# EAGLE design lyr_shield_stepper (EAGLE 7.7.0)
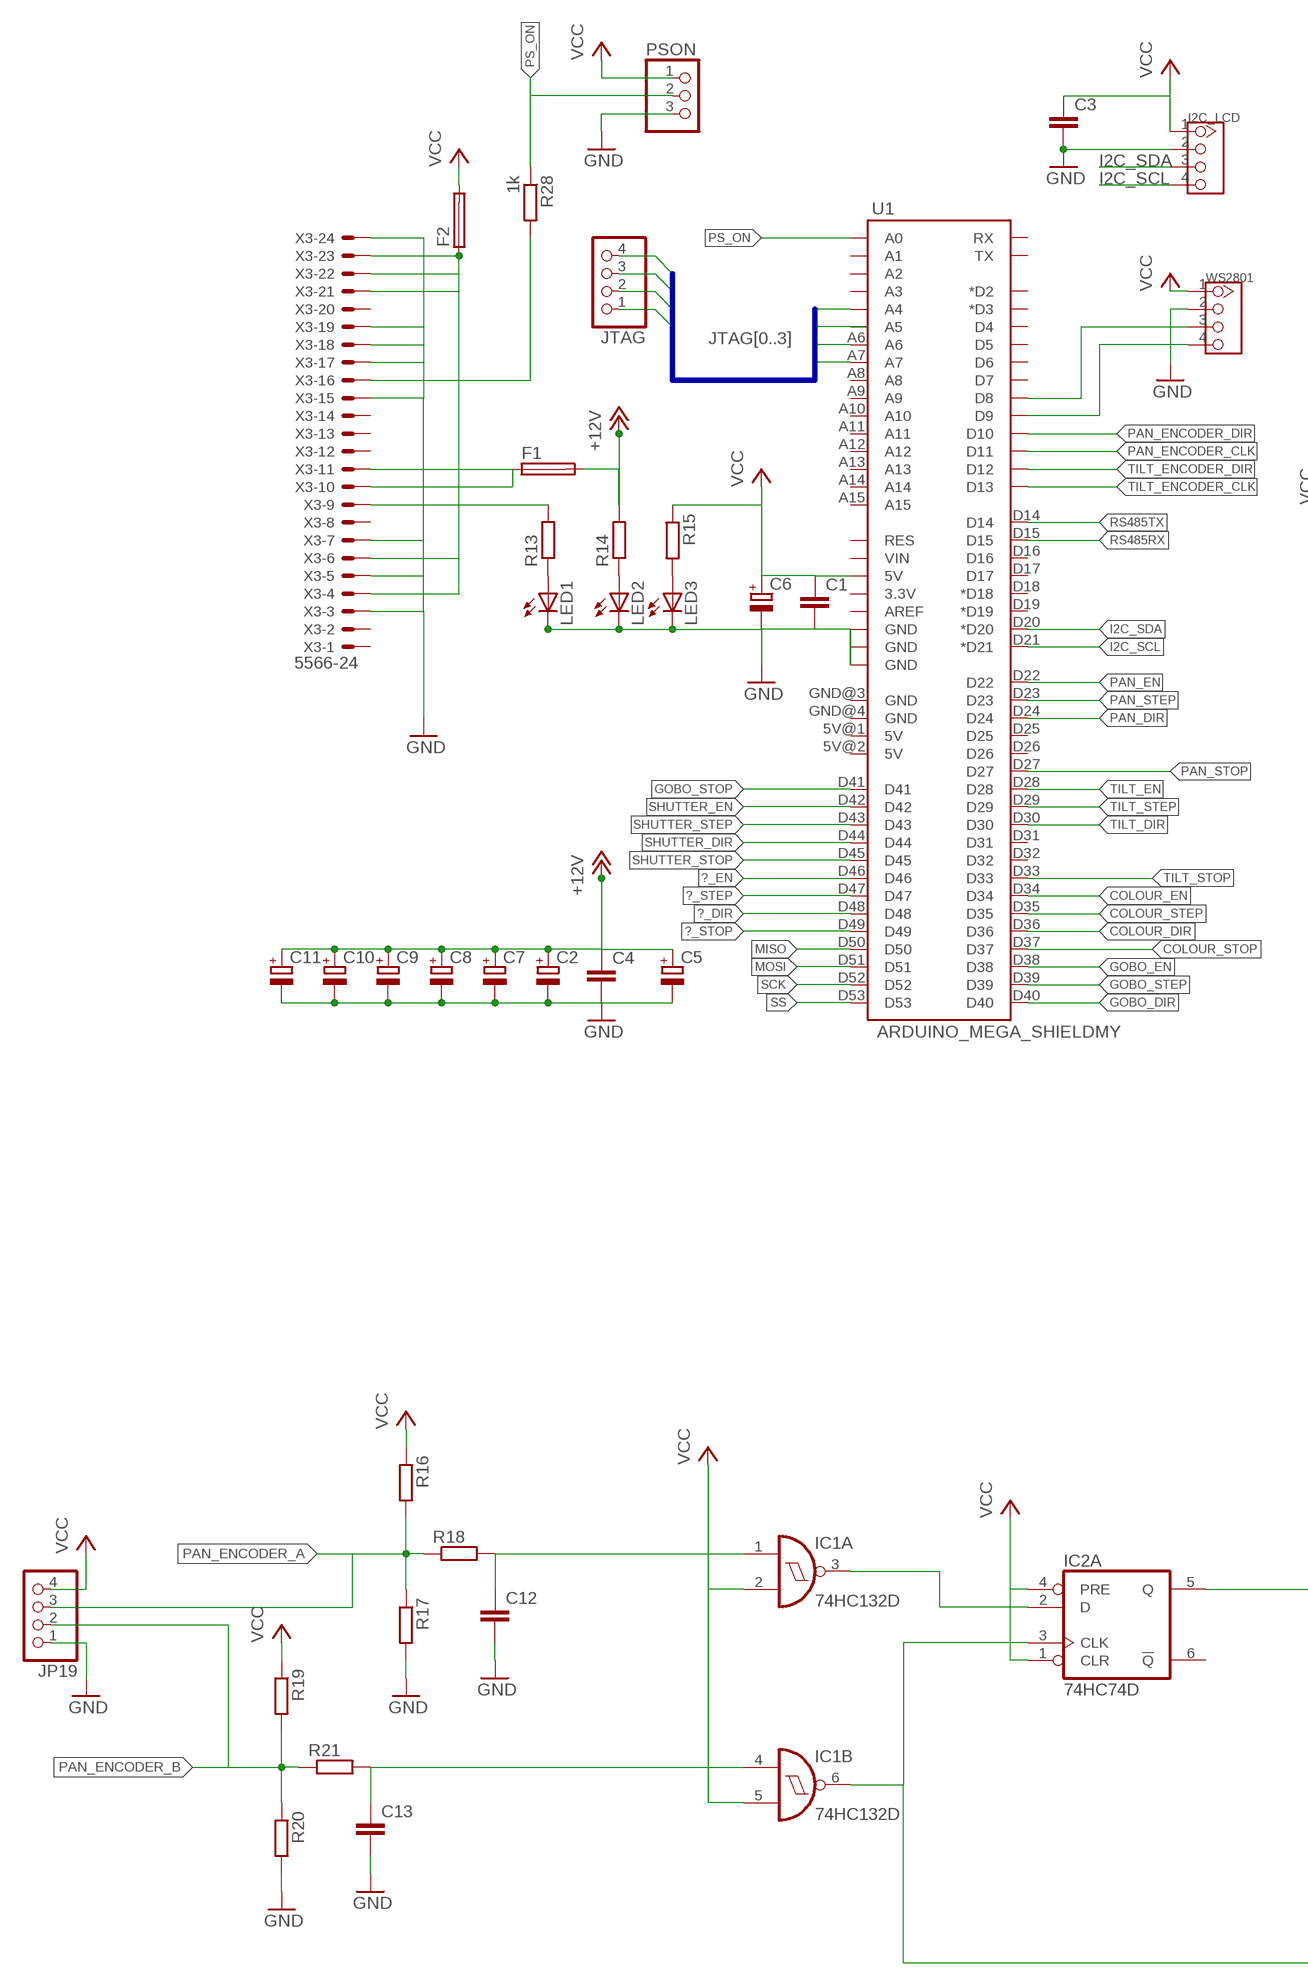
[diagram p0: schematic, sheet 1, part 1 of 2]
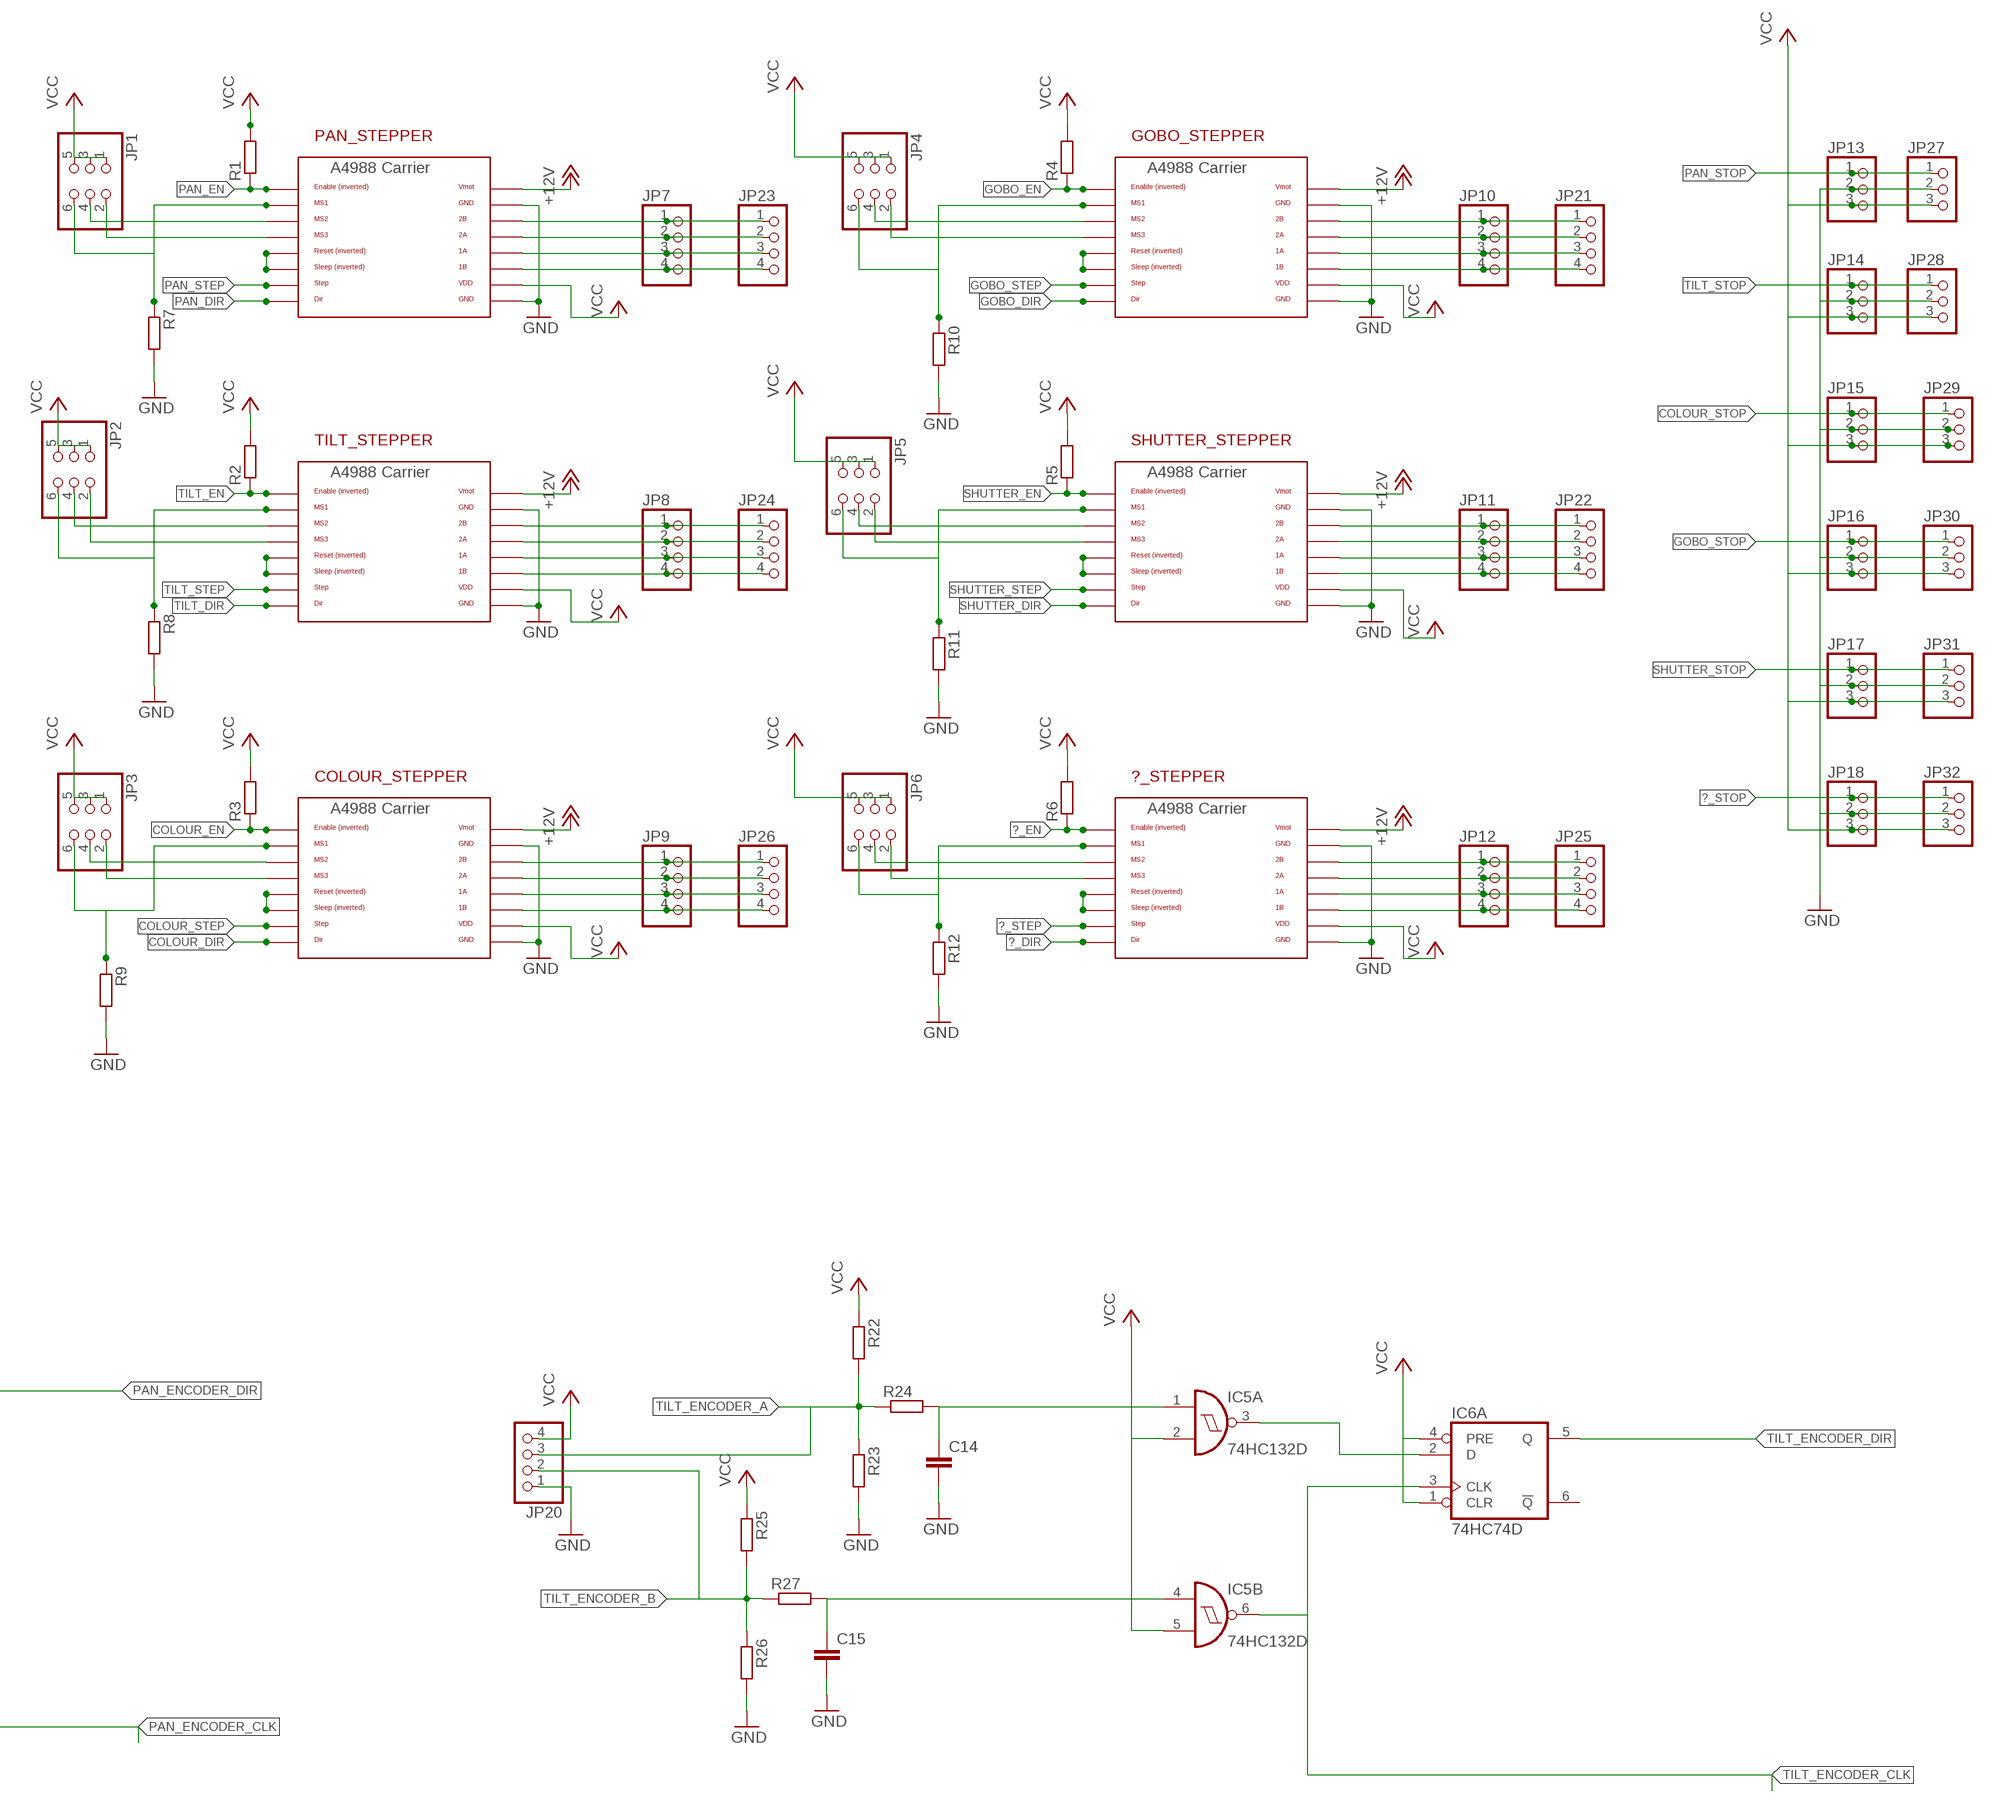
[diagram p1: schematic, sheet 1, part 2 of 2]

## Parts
?_STEPPER  POLOLU_A4983CARRIER  [A4988BREAKOUT]
C1  C-EU025-025X050  [C025-025X050]
C2  CPOL-EUE1.8-4  [E1,8-4]
C3  C-EU025-025X050  [C025-025X050]
C4  C-EU050-025X075  [C050-025X075]
C5  CPOL-EUE5-8.5  [E5-8,5]
C6  CPOL-EUE5-8.5  [E5-8,5]
C7  CPOL-EUE1.8-4  [E1,8-4]
C8  CPOL-EUE1.8-4  [E1,8-4]
C9  CPOL-EUE1.8-4  [E1,8-4]
C10  CPOL-EUE1.8-4  [E1,8-4]
C11  CPOL-EUE1.8-4  [E1,8-4]
C12  C-EU025-025X050  [C025-025X050]
C13  C-EU025-025X050  [C025-025X050]
C14  C-EU025-025X050  [C025-025X050]
C15  C-EU025-025X050  [C025-025X050]
COLOUR_STEPPER  POLOLU_A4983CARRIER  [A4988BREAKOUT]
F1  PTCFUSE  [LITTLEFUSE]
F2  PTCFUSE  [LITTLEFUSE]
GOBO_STEPPER  POLOLU_A4983CARRIER  [A4988BREAKOUT]
I2C_LCD  CONNECTOR_TWIG-4P-2.090D  [CONNECTOR_4P-2.0-90D]
IC1  74HC132D  [SO14]
IC2  74HC74D  [SO14]
IC5  74HC132D  [SO14]
IC6  74HC74D  [SO14]
JP1  PINHD-2X3  [2X03]
JP2  PINHD-2X3  [2X03]
JP3  PINHD-2X3  [2X03]
JP4  PINHD-2X3  [2X03]
JP5  PINHD-2X3  [2X03]
JP6  PINHD-2X3  [2X03]
JP7  PINHD-1X4  [1X04]
JP8  PINHD-1X4  [1X04]
JP9  PINHD-1X4  [1X04]
JP10  PINHD-1X4  [1X04]
JP11  PINHD-1X4  [1X04]
JP12  PINHD-1X4  [1X04]
JP13  PINHD-1X3  [1X03]
JP14  PINHD-1X3  [1X03]
JP15  PINHD-1X3  [1X03]
JP16  PINHD-1X3  [1X03]
JP17  PINHD-1X3  [1X03]
JP18  PINHD-1X3  [1X03]
JP19  PINHD-1X4  [1X04]
JP20  PINHD-1X4  [1X04]
JP21  PINHD-1X4  [1X04]
JP22  PINHD-1X4  [1X04]
JP23  PINHD-1X4  [1X04]
JP24  PINHD-1X4  [1X04]
JP25  PINHD-1X4  [1X04]
JP26  PINHD-1X4  [1X04]
JP27  PINHD-1X3  [1X03]
JP28  PINHD-1X3  [1X03]
JP29  PINHD-1X3  [1X03]
JP30  PINHD-1X3  [1X03]
JP31  PINHD-1X3  [1X03]
JP32  PINHD-1X3  [1X03]
JTAG  PINHD-1X4  [1X04]
LED1  LED5MM  [LED5MM]
LED2  LED5MM  [LED5MM]
LED3  LED5MM  [LED5MM]
PAN_STEPPER  POLOLU_A4983CARRIER  [A4988BREAKOUT]
PSON  PINHD-1X3  [1X03]
R1  R-EU_0207/7  [0207/7]
R2  R-EU_0207/7  [0207/7]
R3  R-EU_0207/7  [0207/7]
R4  R-EU_0207/7  [0207/7]
R5  R-EU_0207/7  [0207/7]
R6  R-EU_0207/7  [0207/7]
R7  R-EU_0207/7  [0207/7]
R8  R-EU_0207/7  [0207/7]
R9  R-EU_0207/7  [0207/7]
R10  R-EU_0207/7  [0207/7]
R11  R-EU_0207/7  [0207/7]
R12  R-EU_0207/7  [0207/7]
R13  R-EU_0207/2V  [0207/2V]
R14  R-EU_0207/2V  [0207/2V]
R15  R-EU_0207/2V  [0207/2V]
R16  R-EU_0207/7  [0207/7]
R17  R-EU_0207/7  [0207/7]
R18  R-EU_0207/7  [0207/7]
R19  R-EU_0207/7  [0207/7]
R20  R-EU_0207/7  [0207/7]
R21  R-EU_0207/7  [0207/7]
R22  R-EU_0207/7  [0207/7]
R23  R-EU_0207/7  [0207/7]
R24  R-EU_0207/7  [0207/7]
R25  R-EU_0207/7  [0207/7]
R26  R-EU_0207/7  [0207/7]
R27  R-EU_0207/7  [0207/7]
R28  1k  R-EU_0207/7  [0207/7]
SHUTTER_STEPPER  POLOLU_A4983CARRIER  [A4988BREAKOUT]
TILT_STEPPER  POLOLU_A4983CARRIER  [A4988BREAKOUT]
U1  ARDUINO_MEGA_SHIELDMY  [MY_ARDUINO_MEGA_SHIELD]
WS2801  CONNECTOR_TWIG-4P-2.090D  [CONNECTOR_4P-2.0-90D]
X3  5566-24  [5566-24]

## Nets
+12V [vcc]: ?_STEPPER.VMOT C2.+ C4.1 C5.+ C7.+ C8.+ C9.+ C10.+ C11.+ COLOUR_STEPPER.VMOT F1.2 GOBO_STEPPER.VMOT PAN_STEPPER.VMOT R14.2 SHUTTER_STEPPER.VMOT TILT_STEPPER.VMOT
?_DIR: ?_STEPPER.DIR U1.D48
?_EN: ?_STEPPER.EN R6.1 U1.D46
?_STEP: ?_STEPPER.STEP U1.D47
?_STOP: JP18.1 JP32.1 U1.D49
COLOUR_DIR: COLOUR_STEPPER.DIR U1.D36
COLOUR_EN: COLOUR_STEPPER.EN R3.1 U1.D34
COLOUR_STEP: COLOUR_STEPPER.STEP U1.D35
COLOUR_STOP: JP15.1 JP29.1 U1.D37
GND [gnd]: ?_STEPPER.GND ?_STEPPER.GND@0(GND) C1.2 C2.- C3.2 C4.2 C5.- C6.- C7.- C8.- C9.- C10.- C11.- C12.2 C13.2 C14.2 C15.2 COLOUR_STEPPER.GND COLOUR_STEPPER.GND@0(GND) GOBO_STEPPER.GND GOBO_STEPPER.GND@0(GND) I2C_LCD.2 JP13.2 JP14.2 JP15.2 JP16.2 JP17.2 JP18.2 JP19.1 JP20.1 JP27.2 JP28.2 JP29.2 JP30.2 JP31.2 JP32.2 LED1.K(C) LED2.K(C) LED3.K(C) PAN_STEPPER.GND PAN_STEPPER.GND@0(GND) PSON.3 R7.2 R8.2 R9.2 R10.2 R11.2 R12.2 R17.2 R20.2 R23.2 R26.2 SHUTTER_STEPPER.GND SHUTTER_STEPPER.GND@0(GND) TILT_STEPPER.GND TILT_STEPPER.GND@0(GND) U1.GND@0(GND) U1.GND@1(GND) U1.GND@2(GND) WS2801.2 X3.3 X3.5 X3.7 X3.15 X3.17 X3.18 X3.19 X3.24
GOBO_DIR: GOBO_STEPPER.DIR U1.D40
GOBO_EN: GOBO_STEPPER.EN R4.1 U1.D38
GOBO_STEP: GOBO_STEPPER.STEP U1.D39
GOBO_STOP: JP16.1 JP30.1 U1.D41
I2C_SCL: I2C_LCD.4 U1.D21(*D21)
I2C_SDA: I2C_LCD.3 U1.D20(*D20)
JTAG0: JTAG.1 U1.A4
JTAG1: JTAG.2
JTAG2: JTAG.3 U1.A6
JTAG3: JTAG.4 U1.A7
MISO: U1.D50
MOSI: U1.D51
N$1: PAN_STEPPER.RST PAN_STEPPER.SLP(SLEEP)
N$2: TILT_STEPPER.RST TILT_STEPPER.SLP(SLEEP)
N$3: COLOUR_STEPPER.RST COLOUR_STEPPER.SLP(SLEEP)
N$4: GOBO_STEPPER.RST GOBO_STEPPER.SLP(SLEEP)
N$5: SHUTTER_STEPPER.RST SHUTTER_STEPPER.SLP(SLEEP)
N$6: ?_STEPPER.RST ?_STEPPER.SLP(SLEEP)
N$7: JP1.6 PAN_STEPPER.MS1 R7.1
N$8: JP1.2 PAN_STEPPER.MS3
N$9: JP1.4 PAN_STEPPER.MS2
N$10: JP2.6 R8.1 TILT_STEPPER.MS1
N$11: JP2.2 TILT_STEPPER.MS3
N$12: JP2.4 TILT_STEPPER.MS2
N$13: COLOUR_STEPPER.MS1 JP3.6 R9.1
N$14: COLOUR_STEPPER.MS3 JP3.2
N$15: COLOUR_STEPPER.MS2 JP3.4
N$16: GOBO_STEPPER.MS1 JP4.6 R10.1
N$17: GOBO_STEPPER.MS3 JP4.2
N$18: GOBO_STEPPER.MS2 JP4.4
N$19: JP5.6 R11.1 SHUTTER_STEPPER.MS1
N$20: JP5.2 SHUTTER_STEPPER.MS3
N$21: JP5.4 SHUTTER_STEPPER.MS2
N$22: ?_STEPPER.MS1 JP6.6 R12.1
N$23: ?_STEPPER.MS3 JP6.2
N$24: ?_STEPPER.MS2 JP6.4
N$25 [vcc]: JP7.1 JP23.1 PAN_STEPPER.2B
N$26 [vcc]: JP7.2 JP23.2 PAN_STEPPER.2A
N$27 [vcc]: JP7.3 JP23.3 PAN_STEPPER.1A
N$28: IC1.3(A:O) IC2.2(A:D)
N$29: C12.1 IC1.1(A:I0) R18.2
N$30: R28.2 X3.16
N$31 [vcc]: JP7.4 JP23.4 PAN_STEPPER.1B
N$32 [vcc]: JP8.1 JP24.1 TILT_STEPPER.2B
N$33 [vcc]: JP8.2 JP24.2 TILT_STEPPER.2A
N$34 [vcc]: JP8.3 JP24.3 TILT_STEPPER.1A
N$35 [vcc]: JP8.4 JP24.4 TILT_STEPPER.1B
N$36 [vcc]: COLOUR_STEPPER.2B JP9.1 JP26.1
N$37 [vcc]: COLOUR_STEPPER.2A JP9.2 JP26.2
N$38 [vcc]: COLOUR_STEPPER.1A JP9.3 JP26.3
N$39 [vcc]: COLOUR_STEPPER.1B JP9.4 JP26.4
N$40 [vcc]: GOBO_STEPPER.2B JP10.1 JP21.1
N$41 [vcc]: GOBO_STEPPER.2A JP10.2 JP21.2
N$42 [vcc]: GOBO_STEPPER.1A JP10.3 JP21.3
N$43 [vcc]: GOBO_STEPPER.1B JP10.4 JP21.4
N$44 [vcc]: JP11.1 JP22.1 SHUTTER_STEPPER.2B
N$45 [vcc]: JP11.2 JP22.2 SHUTTER_STEPPER.2A
N$46 [vcc]: JP11.3 JP22.3 SHUTTER_STEPPER.1A
N$47 [vcc]: JP11.4 JP22.4 SHUTTER_STEPPER.1B
N$48 [vcc]: ?_STEPPER.2B JP12.1 JP25.1
N$49 [vcc]: ?_STEPPER.2A JP12.2 JP25.2
N$50 [vcc]: ?_STEPPER.1A JP12.3 JP25.3
N$51 [vcc]: ?_STEPPER.1B JP12.4 JP25.4
N$52: LED1.A R13.1
N$53: U1.D8 WS2801.3
N$54: R13.2 X3.9
N$55: LED3.A R15.2
N$56: LED2.A R14.1
N$57: U1.D9 WS2801.4
N$58 [vcc]: F1.1 X3.10 X3.11
N$60 [vcc]: F2.1 X3.4 X3.6 X3.21 X3.22 X3.23
N$61: C13.1 IC1.4(B:I0) R21.2
N$62: IC5.3(A:O) IC6.2(A:D)
N$63: C14.1 IC5.1(A:I0) R24.2
N$64: C15.1 IC5.4(B:I0) R27.2
PAN_DIR: PAN_STEPPER.DIR U1.D24
PAN_EN: PAN_STEPPER.EN R1.1 U1.D22
PAN_ENCODER_A: JP19.3 R16.2 R17.1 R18.1
PAN_ENCODER_B: JP19.2 R19.2 R20.1 R21.1
PAN_ENCODER_CLK: IC1.6(B:O) IC2.3(A:CLK)
PAN_ENCODER_DIR: IC2.5(A:Q)
PAN_STEP: PAN_STEPPER.STEP U1.D23
PAN_STOP: JP13.1 JP27.1 U1.D27
PS_ON: PSON.2 R28.1
RS485RX: U1.D15
RS485TX: U1.D14
SCK: U1.D52
SHUTTER_DIR: SHUTTER_STEPPER.DIR U1.D44
SHUTTER_EN: R5.1 SHUTTER_STEPPER.EN U1.D42
SHUTTER_STEP: SHUTTER_STEPPER.STEP U1.D43
SHUTTER_STOP: JP17.1 JP31.1 U1.D45
SS: U1.D53
TILT_DIR: TILT_STEPPER.DIR U1.D30
TILT_EN: R2.1 TILT_STEPPER.EN U1.D28
TILT_ENCODER_A: JP20.3 R22.2 R23.1 R24.1
TILT_ENCODER_B: JP20.2 R25.2 R26.1 R27.1
TILT_ENCODER_CLK: IC5.6(B:O) IC6.3(A:CLK)
TILT_ENCODER_DIR: IC6.5(A:Q)
TILT_STEP: TILT_STEPPER.STEP U1.D29
TILT_STOP: JP14.1 JP28.1 U1.D33
VCC [vcc]: ?_STEPPER.VDD C1.1 C3.1 C6.+ COLOUR_STEPPER.VDD F2.2 GOBO_STEPPER.VDD I2C_LCD.1 IC1.2(A:I1) IC1.5(B:I1) IC2.1(A:CLR) IC2.4(A:PRE) IC5.2(A:I1) IC5.5(B:I1) IC6.1(A:CLR) IC6.4(A:PRE) JP1.1 JP1.3 JP1.5 JP2.1 JP2.3 JP2.5 JP3.1 JP3.3 JP3.5 JP4.1 JP4.3 JP4.5 JP5.1 JP5.3 JP5.5 JP6.1 JP6.3 JP6.5 JP13.3 JP14.3 JP15.3 JP16.3 JP17.3 JP18.3 JP19.4 JP20.4 JP27.3 JP28.3 JP29.3 JP30.3 JP31.3 JP32.3 PAN_STEPPER.VDD PSON.1 R1.2 R2.2 R3.2 R4.2 R5.2 R6.2 R15.1 R16.1 R19.1 R22.1 R25.1 SHUTTER_STEPPER.VDD TILT_STEPPER.VDD U1.5V@0(5V) WS2801.1
Unconnected: IC1.8(C:O) IC1.9(C:I0) IC1.10(C:I1) IC1.11(D:O) IC1.12(D:I0) IC1.13(D:I1) IC2.6(A:!Q) IC2.8(B:!Q) IC2.9(B:Q) IC2.10(B:PRE) IC2.11(B:CLK) IC2.12(B:D) IC2.13(B:CLR) IC5.8(C:O) IC5.9(C:I0) IC5.10(C:I1) IC5.11(D:O) IC5.12(D:I0) IC5.13(D:I1) IC6.6(A:!Q) IC6.8(B:!Q) IC6.9(B:Q) IC6.10(B:PRE) IC6.11(B:CLK) IC6.12(B:D) IC6.13(B:CLR) U1.3.3V U1.5V@1(5V) U1.5V@2(5V) U1.A0 U1.A1 U1.A2 U1.A3 U1.A5 U1.A8 U1.A9 U1.A10 U1.A11 U1.A12 U1.A13 U1.A14 U1.A15 U1.AREF U1.D2(*D2) U1.D3(*D3) U1.D4 U1.D5 U1.D6 U1.D7 U1.D10 U1.D11 U1.D12 U1.D13 U1.D16 U1.D17 U1.D18(*D18) U1.D19(*D19) U1.D25 U1.D26 U1.D31 U1.D32 U1.GND@3(GND) U1.GND@4(GND) U1.RES U1.RX U1.TX U1.VIN X3.1 X3.2 X3.8 X3.12 X3.13 X3.14 X3.20

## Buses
JTAG[0..3]

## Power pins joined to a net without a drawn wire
GND: IC1.7(P:GND) IC2.7(P:GND) IC5.7(P:GND) IC6.7(P:GND)
VCC: IC1.14(P:VCC) IC2.14(P:VCC) IC5.14(P:VCC) IC6.14(P:VCC)

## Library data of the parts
?_STEPPER COLOUR_STEPPER GOBO_STEPPER PAN_STEPPER SHUTTER_STEPPER TILT_STEPPER = lyr_shield_stepper:POLOLU_A4983CARRIER
C1 C3 C4 C12-C15 = rcl:C-EU: CAPACITOR, European symbol
C2 C5-C11 = rcl:CPOL-EU: POLARIZED CAPACITOR, European symbol
F1 F2 = RepRapjr:PTCFUSE: LITTLEFUSE
I2C_LCD WS2801 = lyr_shield_stepper:CONNECTOR_TWIG-4P-2.0
IC1 IC5 = 74xx-eu:74*132: Quad 2-input NAND schmitt trigger
IC2 IC6 = 74xx-eu:74*74: Dual D type positive edge triggered FLIP FLOP, preset and clear
JP1-JP6 = pinhead:PINHD-2X3: PIN HEADER
JP7-JP12 JP19-JP26 JTAG = pinhead:PINHD-1X4: PIN HEADER
JP13-JP18 JP27-JP32 PSON = pinhead:PINHD-1X3: PIN HEADER
LED1-LED3 = RepRapjr:LED: LED
R1-R28 = rcl:R-EU_: RESISTOR, European symbol
U1 = RepRapjr:ARDUINO_MEGA_SHIELD
X3 = con-molex:5566-24: Mini FIT connector 24 pol Source: http://www.molex.com; OC_FARNELL: unknown; OC_NEWARK: unknown

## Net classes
0 default: width 0.406 mm
1 vcc: width 0.813 mm
2 gnd: width 0.813 mm

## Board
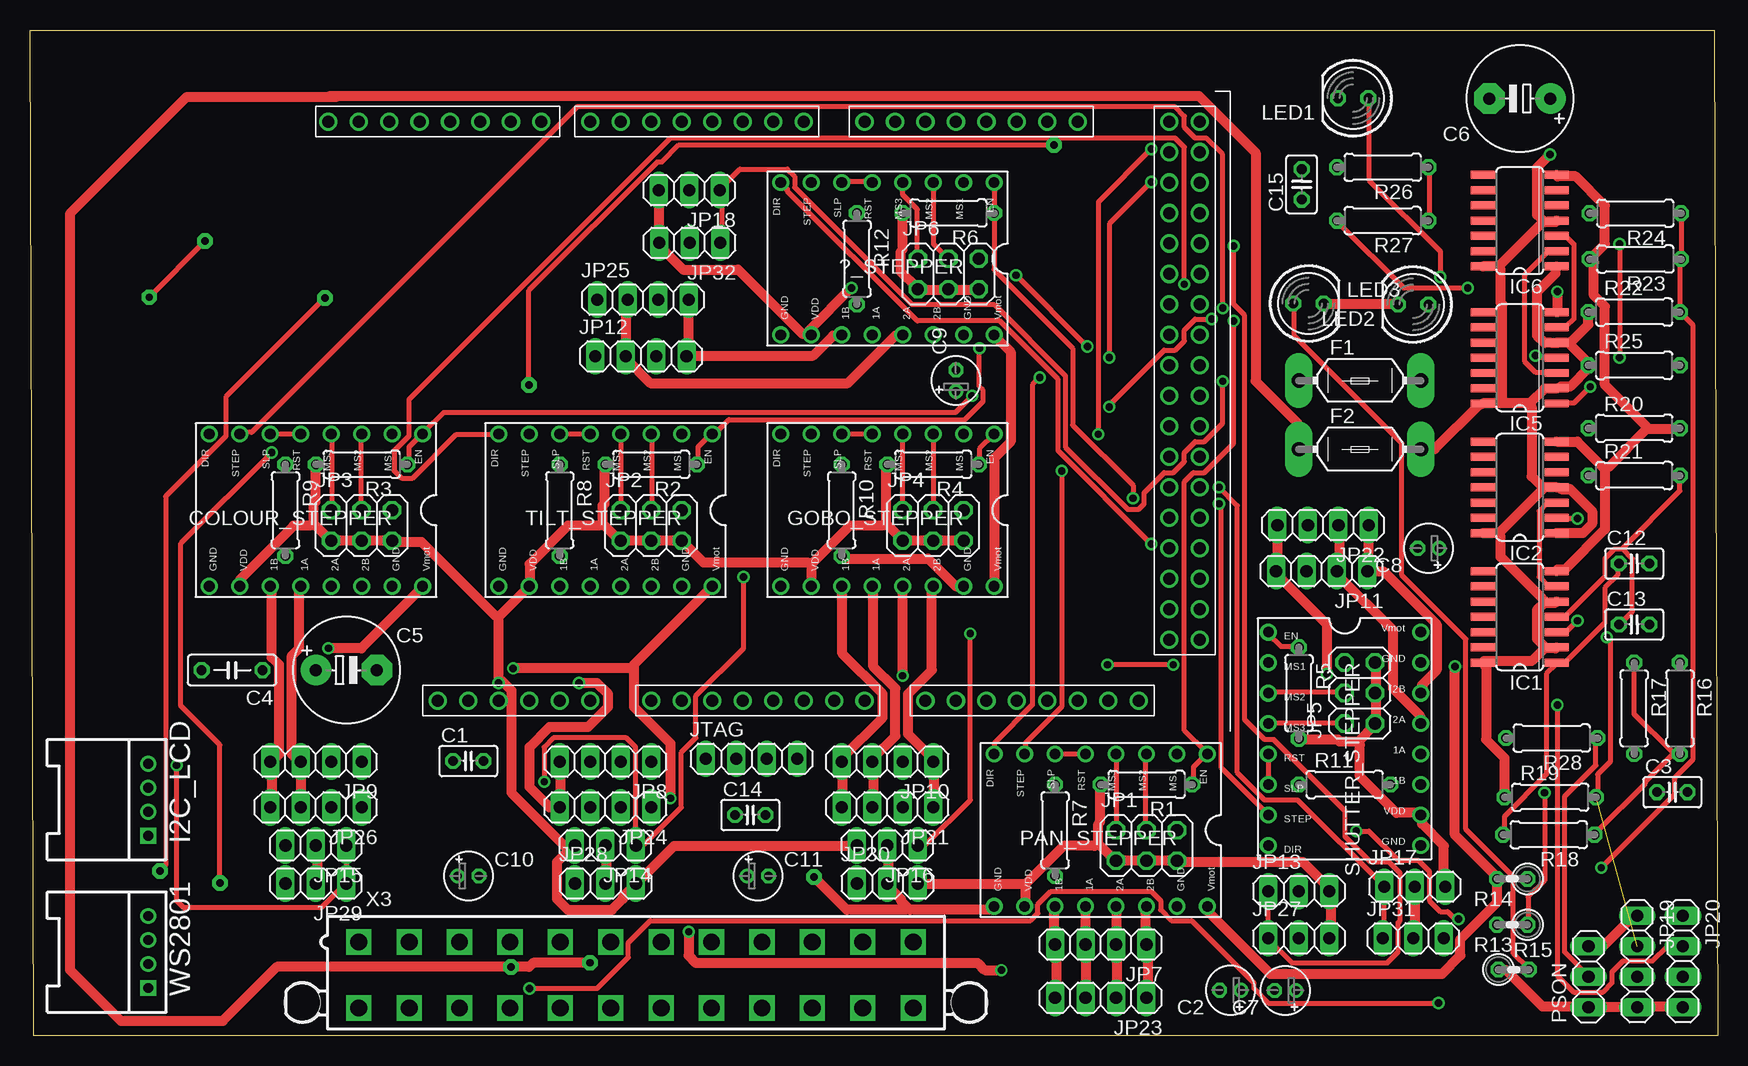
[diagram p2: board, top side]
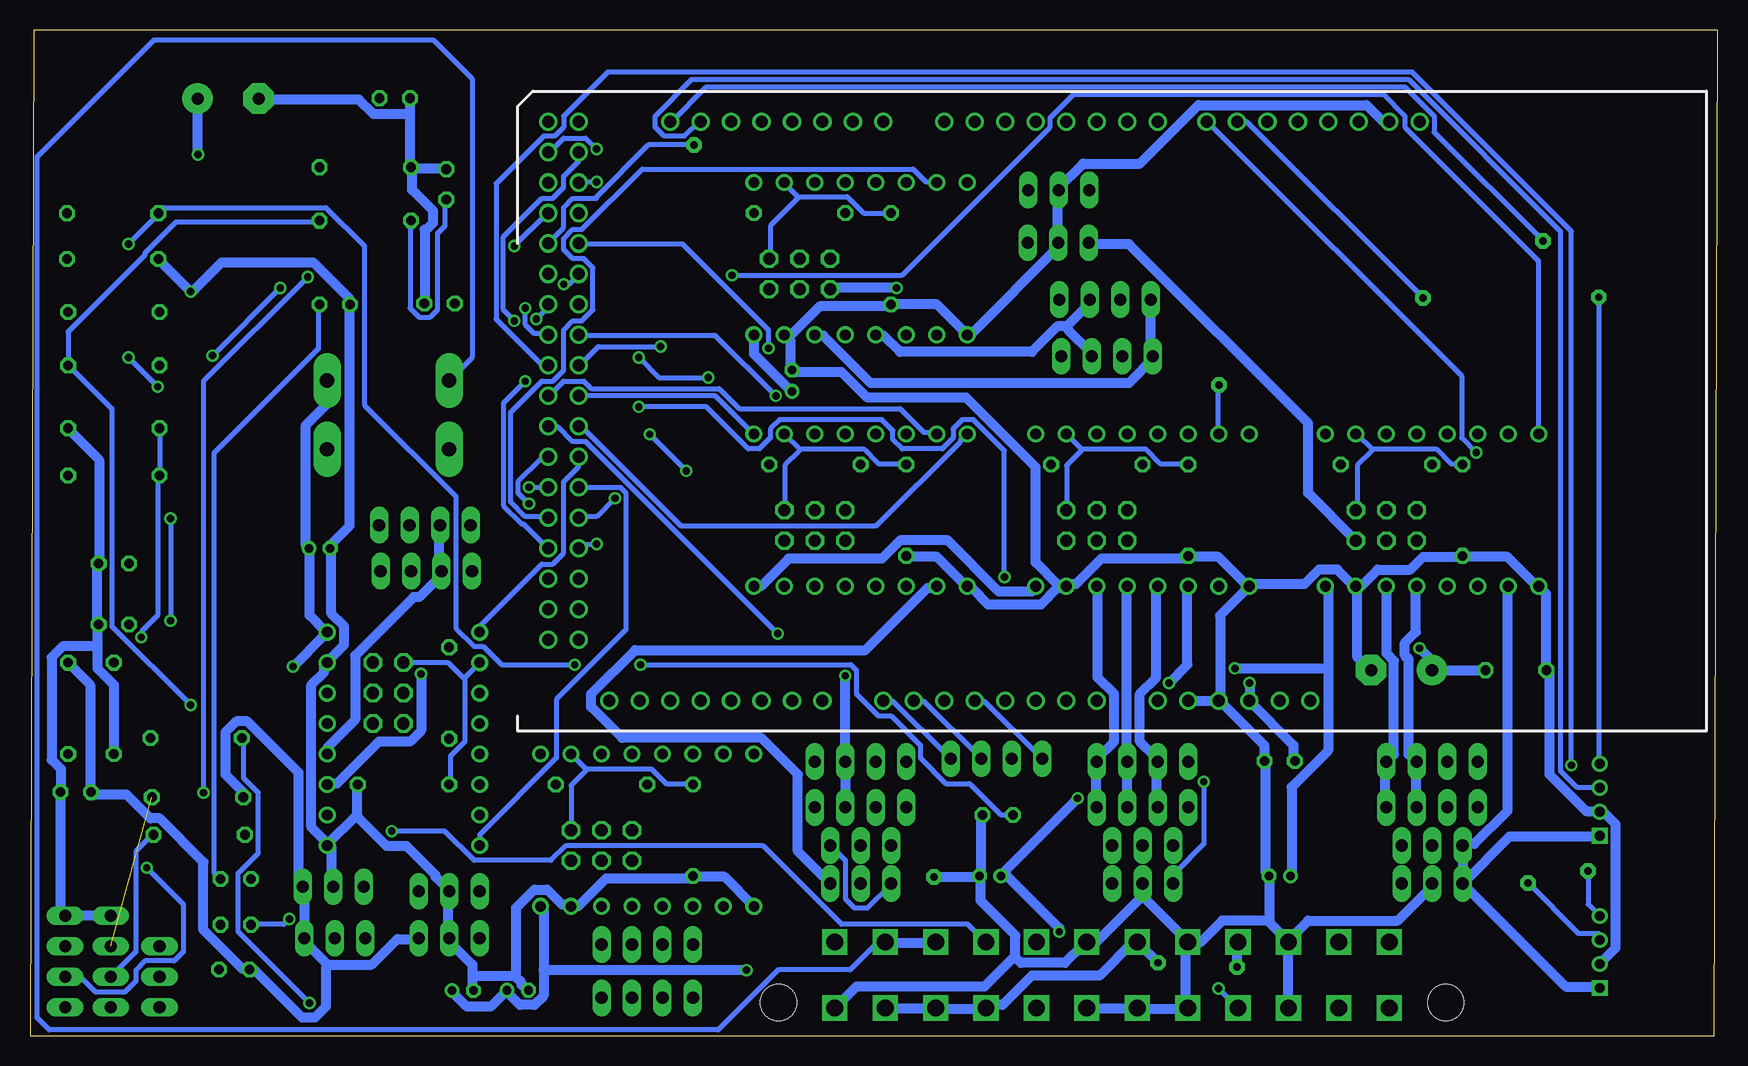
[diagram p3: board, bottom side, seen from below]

Size 140.67 x 83.83 mm. Coordinates in mm from the lower left corner, seen from the top.
Outline: 0.33,0 0,83.82 140.36,83.83 140.67,0.01 0.33,0
Copper layers (1*16): Top 0.035mm / dielectric 1.5mm / Bottom 0.035mm
Design rules "default": minimum track width 10mil, minimum drill 24mil, track to track 8mil, track to pad 8mil, pad to pad 8mil, via to via 8mil, smd to smd 8mil, copper to edge 40mil, drill to drill 8mil, minimum pad ring 10mil, minimum via ring 8mil, stop-mask expansion 4mil, vias tented up to drill 0mil, thermal gap 10mil
tRestrict: area 51.1,27.3 to 52.4,28.6; area 43.5,27.3 to 44.8,28.6; area 41,27.3 to 42.2,28.6; area 46,27.3 to 47.3,28.6; area 61.3,27.3 to 62.6,28.6; area 66.4,27.3 to 67.6,28.6; area 68.9,27.3 to 70.2,28.6; area 96.8,47.6 to 98.1,48.9; area 96.8,40 to 98.1,41.3; area 94.3,40 to 95.6,41.3; area 94.3,42.5 to 95.6,43.8; area 96.8,42.5 to 98.1,43.8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

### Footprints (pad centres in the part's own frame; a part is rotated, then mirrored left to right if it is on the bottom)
A4988BREAKOUT = drill 0.9: 1A 8.89,1.27; 1B 11.43,1.27; 2A 6.35,1.27; 2B 3.81,1.27; DIR 16.51,-11.43; EN -1.27,-11.43; GND 16.51,1.27; GND@0 1.27,1.27; MS1 1.27,-11.43; MS2 3.81,-11.43; MS3 6.35,-11.43; RST 8.89,-11.43; SLP 11.43,-11.43; STEP 13.97,-11.43; VDD 13.97,1.27; VMOT -1.27,1.27
C025-025X050 = drill 0.813 octagon: 1 -1.27,0; 2 1.27,0
E1,8-4 = drill 0.711 pad 1.168: + -0.889,0 | drill 0.711 pad 1.168 octagon: - 0.889,0
C050-025X075 = drill 0.813 octagon: 1 -2.54,0; 2 2.54,0
E5-8,5 = drill 1.016 pad 2.54: + -2.54,0 | drill 1.016 pad 2.54 octagon: - 2.54,0
LITTLEFUSE = drill 1.2 pad 2.3 long: 1 -5.08,0; 2 5.08,0
CONNECTOR_4P-2.0-90D = drill 0.8 pad 1.27 square: 1 -3,0 | drill 0.8 pad 1.27: 2 -1,0; 3 1,0; 4 3,0
SO14 = smd 0.66 x 2.032: 1 -3.81,-3.073; 2 -2.54,-3.073; 3 -1.27,-3.073; 4 0,-3.073; 5 1.27,-3.073; 6 2.54,-3.073; 7 3.81,-3.073; 8 3.81,3.073; 9 2.54,3.073; 10 1.27,3.073; 11 0,3.073; 12 -1.27,3.073; 13 -2.54,3.073; 14 -3.81,3.073
2X03 = drill 1.016 octagon: 1 -2.54,-1.27; 2 -2.54,1.27; 3 0,-1.27; 4 0,1.27; 5 2.54,-1.27; 6 2.54,1.27
1X04 = drill 1.016 long: 1 -3.81,0; 2 -1.27,0; 3 1.27,0; 4 3.81,0
1X03 = drill 1.016 long: 1 -2.54,0; 2 0,0; 3 2.54,0
LED5MM = drill 0.813 octagon: A -1.27,0; K 1.27,0
0207/7 = drill 0.813 octagon: 1 -3.81,0; 2 3.81,0
0207/2V = drill 0.813 octagon: 1 -1.27,0; 2 1.27,0
MY_ARDUINO_MEGA_SHIELD = drill 1 pad 1.422: 3.3V 63.5,50.8; 5V@0 60.96,50.8; 5V@1 5.08,2.54; 5V@2 2.54,2.54; A0 48.26,50.8; A1 45.72,50.8; A2 43.18,50.8; A3 40.64,50.8; A4 38.1,50.8; A5 35.56,50.8; A6 33.02,50.8; A7 30.48,50.8; A8 25.4,50.8; A9 22.86,50.8; A10 20.32,50.8; A11 17.78,50.8; A12 15.24,50.8; A13 12.7,50.8; A14 10.16,50.8; A15 7.62,50.8; AREF 75.184,2.54; D2 40.64,2.54; D3 43.18,2.54; D4 45.72,2.54; D5 48.26,2.54; D6 50.8,2.54; D7 53.34,2.54; D8 57.404,2.54; D9 59.944,2.54; D10 62.484,2.54; D11 65.024,2.54; D12 67.564,2.54; D13 70.104,2.54; D14 30.48,2.54; D15 27.94,2.54; D16 25.4,2.54; D17 22.86,2.54; D18 20.32,2.54; D19 17.78,2.54; D20 15.24,2.54; D21 12.7,2.54; D22 5.08,5.08; D23 2.54,5.08; D24 5.08,7.62; D25 2.54,7.62; D26 5.08,10.16; D27 2.54,10.16; D28 5.08,12.7; D29 2.54,12.7; D30 5.08,15.24; D31 2.54,15.24; D32 5.08,17.78; D33 2.54,17.78; D34 5.08,20.32; D35 2.54,20.32; D36 5.08,22.86; D37 2.54,22.86; D38 5.08,25.4; D39 2.54,25.4; D40 5.08,27.94; D41 2.54,27.94; D42 5.08,30.48; D43 2.54,30.48; D44 5.08,33.02; D45 2.54,33.02; D46 5.08,35.56; D47 2.54,35.56; D48 5.08,38.1; D49 2.54,38.1; D50 5.08,40.64; D51 2.54,40.64; D52 5.08,43.18; D53 2.54,43.18; GND@0 58.42,50.8; GND@1 55.88,50.8; GND@2 72.644,2.54; GND@3 5.08,45.72; GND@4 2.54,45.72; RES 66.04,50.8; RX 35.56,2.54; TX 38.1,2.54; VIN 53.34,50.8
5566-24 = drill 1.4 square: 1 23.1,-2.75; 2 18.9,-2.75; 3 14.7,-2.75; 4 10.5,-2.75; 5 6.3,-2.75; 6 2.1,-2.75; 7 -2.1,-2.75; 8 -6.3,-2.75; 9 -10.5,-2.75; 10 -14.7,-2.75; 11 -18.9,-2.75; 12 -23.1,-2.75; 13 23.1,2.75; 14 18.9,2.75; 15 14.7,2.75; 16 10.5,2.75; 17 6.3,2.75; 18 2.1,2.75; 19 -2.1,2.75; 20 -6.3,2.75; 21 -10.5,2.75; 22 -14.7,2.75; 23 -18.9,2.75; 24 -23.1,2.75 | hole 3: 27.8,2.29; -27.8,2.29

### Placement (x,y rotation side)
?_STEPPER  79.07,59.69 180 top
C1  36.52,22.91 0 top
C2  100.02,3.81 180 top
C3  136.86,20.32 0 top
C4  16.84,30.48 180 top
C5  26.36,30.48 0 top
C6  124.16,78.11 180 top
C7  104.61,3.79 180 top
C8  116.53,40.64 180 top
C9  77.16,54.61 90 top
C10  36.52,13.34 0 top
C11  60.66,13.34 0 top
C12  133.68,39.37 0 top
C13  133.68,34.29 0 top
C14  60.02,18.41 0 top
C15  105.97,70.97 90 top
COLOUR_STEPPER  31.44,38.73 180 top
F1  110.82,54.61 0 top
F2  110.82,48.9 0 top
GOBO_STEPPER  79.07,38.73 180 top
I2C_LCD  9.86,19.68 90 top
IC1  124.16,34.92 90 top
IC2  124.16,45.72 90 top
IC5  124.16,56.52 90 top
IC6  124.16,67.94 90 top
JP1  93.04,15.88 0 top
JP2  51.77,42.55 0 top
JP3  27.63,42.55 0 top
JP4  75.26,42.55 0 top
JP5  110.82,28.57 90 top
JP6  76.53,63.5 0 top
JP7  89.23,7.62 180 top
JP8  47.95,22.86 180 top
JP9  23.82,22.86 180 top
JP10  71.45,22.86 180 top
JP11  107.64,38.73 180 top
JP12  50.91,56.64 0 top
JP13  105.74,12.06 0 top
JP14  47.95,15.88 180 top
JP15  23.82,15.88 180 top
JP16  71.45,15.88 180 top
JP17  115.39,12.44 0 top
JP18  54.94,70.48 180 top
JP19  133.93,6.21 270 top
JP20  137.74,6.21 270 top
JP21  71.45,19.05 180 top
JP22  107.77,42.57 180 top
JP23  89.23,3.17 180 top
JP24  47.95,19.05 180 top
JP25  51.07,61.36 0 top
JP26  23.82,19.05 180 top
JP27  105.74,8.14 0 top
JP28  47.95,12.7 0 top
JP29  23.82,12.7 180 top
JP30  71.45,12.7 0 top
JP31  115.27,8.14 0 top
JP32  54.97,66.09 180 top
JTAG  60.12,23.09 0 top
LED1  110.27,78.14 180 top
LED2  115.27,60.96 180 top
LED3  106.53,61.04 0 top
PAN_STEPPER  96.85,12.06 180 top
PSON  129.87,4.95 90 top
R1  93.04,20.95 180 top
R2  51.77,47.62 180 top
R3  27.63,47.62 180 top
R4  75.26,47.62 180 top
R5  105.74,28.57 270 top
R6  76.53,68.58 180 top
R7  85.42,17.14 270 top
R8  44.14,43.81 270 top
R9  21.28,43.81 270 top
R10  67.64,43.81 270 top
R11  109.55,20.95 0 top
R12  68.91,64.77 270 top
R13  123.52,9.28 180 top
R14  123.52,13.09 180 top
R15  123.64,5.54 0 top
R16  137.49,27.3 270 top
R17  133.68,27.3 270 top
R18  126.56,16.77 180 top
R19  126.69,19.89 0 top
R20  133.68,50.65 0 top
R21  133.68,46.7 0 top
R22  133.68,60.33 0 top
R23  133.78,64.75 180 top
R24  133.78,68.56 180 top
R25  133.68,55.88 0 top
R26  112.72,72.39 180 top
R27  112.72,67.94 180 top
R28  126.81,24.82 180 top
SHUTTER_STEPPER  114.63,32.38 270 top
TILT_STEPPER  55.57,38.73 180 top
U1  100.02,78.74 180 top
WS2801  9.86,6.99 90 top
X3  50.49,5.08 180 top

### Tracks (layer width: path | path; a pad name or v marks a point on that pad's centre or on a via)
+12V  (via drill 0.61)
  Top 0.813: PAN_STEPPER.VMOT 98.17,10.67 98.17,10.36 103.35,5.18 117.68,5.18 119.2,6.71 119.2,8.08 122.25,11.12 R14.2 122.1,13.41 118.75,16.76 v118.75,30.79 | v24.87,32.31 27.61,32.31 32.64,37.34 COLOUR_STEPPER.VMOT | GOBO_STEPPER.VMOT 80.34,48.16 81.71,49.53 81.71,57 80.34,58.37 ?_STEPPER.VMOT | v53.36,19.81 53.36,24.38 50.32,27.43 50.32,30.63 | 50.32,30.63 50.32,30.94 TILT_STEPPER.VMOT | 50.32,30.63 v40.26,30.63 | v80.95,5.49 79.58,5.49 78.97,6.1 55.5,6.1 54.89,6.71 v54.89,8.69
  Bottom 0.813: F1.2 116,54.56 116,52.58 117.68,50.9 117.68,40.84 C8.+ 117.37,40.54 117.37,35.05 116,33.68 SHUTTER_STEPPER.VMOT 116.15,33.38 v118.75,30.79 | C7.+ 105.49,3.66 104.27,2.44 102.29,2.44 C2.+ 100.76,3.5 99.85,2.59 98.63,2.59 97.87,3.35 97.87,5.49 | 97.87,5.49 97.87,10.52 98.02,10.67 PAN_STEPPER.VMOT | C4.1 C5.+ 23.95,30.79 23.95,31.39 v24.87,32.31 | 32.49,30.63 32.49,37.19 32.64,37.34 COLOUR_STEPPER.VMOT | 32.49,30.63 32.49,23.77 35.53,20.73 35.53,13.41 C10.+ | ?_STEPPER.VMOT 80.34,56.84 77.29,53.8 C9.+ | v53.36,19.81 59.77,13.41 C11.+ 59.31,13.41 54.89,8.99 v54.89,8.69 | GOBO_STEPPER.VMOT 80.34,37.49 79.73,37.49 77.44,39.78 69.67,39.78 68.15,41.3 64.19,41.3 59.92,37.03 57.17,37.03 56.87,37.34 TILT_STEPPER.VMOT | v40.26,30.63 32.49,30.63 | v80.95,5.49 97.87,5.49
?_DIR  (via drill 0.61)
  Top 0.406: ?_STEPPER.DIR 63.12,70.56 63.12,70.41 73.94,59.59 80.8,59.59 85.67,54.71 85.67,48.77 v93.45,41
  Bottom 0.406: v93.45,41 94.51,41 94.82,40.69 U1.D48
?_EN  (via drill 0.61)
  Top 0.406: ?_STEPPER.EN R6.1 80.34,63.86 86.89,57.3 86.89,50.9 91.92,45.87 v91.92,44.81
  Bottom 0.406: v91.92,44.81 93.45,43.28 94.82,43.28 U1.D46
?_STEP
  Bottom 0.406: ?_STEPPER.STEP 65.1,71.17 66.01,71.17 67.08,72.24 89.64,72.24 94.67,67.21 95.43,67.21 96.19,66.45 96.19,65.53 95.43,64.77 94.51,64.77 93.75,64.01 93.75,60.5 94.67,59.59 95.43,59.59 96.19,58.83 96.19,55.47 97.1,54.56 98.02,54.56 100.61,51.97 100.61,44.5 99.39,43.28 97.56,43.28 U1.D47
?_STOP  (via drill 0.61)
  Top 0.406: v99.39,54.56 99.39,51.05 97.87,49.53 97.1,49.53 96.19,48.62 96.19,47.85 95.27,46.94 94.51,46.94 92.84,45.26 92.84,44.35 92.38,43.89 91.47,43.89 86.28,49.07 86.28,55.02 80.34,60.96 73.48,60.96 63.73,70.71 63.73,71.63 63.12,72.24 59.16,72.24 57.48,70.56 JP18.1 57.63,70.41 57.63,66.14 JP32.1
  Bottom 0.406: v99.39,54.56 101.22,52.73 101.22,44.2 99.69,42.67 99.54,42.67 97.56,40.69 U1.D49
COLOUR_DIR  (via drill 0.61)
  Top 0.406: v88.11,57.45 v82.17,63.4
  Bottom 0.406: v82.17,63.4 68,63.4 55.65,75.74 55.65,76.5 53.67,78.49 27.91,78.49 26.09,76.66 26.09,75.74 14.96,64.62 14.96,50.29 COLOUR_STEPPER.DIR | v88.11,57.45 93.29,57.45 94.82,55.93 U1.D36
COLOUR_EN  (via drill 0.61)
  Top 0.406: R3.1 31.57,47.7 31.57,49.07 32.64,50.14 COLOUR_STEPPER.EN 32.79,50.29 34.47,51.97 77.14,51.97 v78.51,53.34
  Bottom 0.406: v78.51,53.34 83.54,58.37 94.82,58.37 U1.D34
COLOUR_STEP  (via drill 0.61)
  Top 0.406: v99.39,60.66 99.39,73.46 98.02,74.83 97.1,74.83 96.19,75.74 96.19,76.66 95.43,77.42 45.59,77.42 18.47,50.29 17.55,50.29 COLOUR_STEPPER.STEP
  Bottom 0.406: v99.39,60.66 99.39,59.28 98.63,58.52 97.56,58.52 U1.D35
COLOUR_STOP  (via drill 0.61)
  Top 0.406: v12.22,22.55 12.22,11.28 12.83,10.67 24.26,10.67 26.24,12.65 JP29.1 26.39,12.8 26.39,15.85 JP15.1
  Bottom 0.406: v12.22,22.55 12.22,67.06 25.48,80.31 92.53,80.31 96.19,76.66 96.19,75.74 96.95,74.98 97.87,74.98 101.83,71.02 101.83,59.74 98.02,55.93 97.56,55.93 U1.D37
GND  (via drill 0.6 pad 1.27, 0.61)
  Top 0.813: LED2.K 107.92,60.96 LED3.K | PSON.3 129.87,7.62 131.24,7.62 133.53,9.91 133.83,9.91 JP19.1 | v127.28,62.03 127.28,60.35 IC5.7 | IC6.7 127.28,71.63 128.8,71.63 131.24,69.19 131.24,65.99 130.02,64.77 R23.2 130.33,64.47 130.33,61.72 131.24,60.81 131.24,54.25 134.59,50.9 134.75,50.6 | 131.24,47.24 131.24,42.22 127.89,38.86 127.28,38.86 IC1.7 | 131.24,47.24 128.96,49.53 IC2.7 | 134.75,50.6 137.49,50.6 R20.2 | 134.75,50.6 131.55,47.4 131.24,47.24 | JP16.2 71.5,15.85 71.5,12.8 JP30.2 71.65,12.34 72.57,11.43 72.57,11.28 73.33,10.52 | 73.33,10.52 80.19,10.52 80.34,10.67 PAN_STEPPER.GND | JP31.2 115.39,8.23 115.39,12.34 JP17.2 | JP28.2 48.03,12.8 48.03,15.85 JP14.2 | JP29.2 23.95,12.8 23.95,15.85 JP15.2 | GOBO_STEPPER.GND@0 77.75,37.49 77.14,37.49 74.85,39.78 67.84,39.78 67.69,39.93 R10.2 | 73.33,10.52 68.06,10.52 v65.33,13.25
  Bottom 0.813: 108.84,72.39 R26.2 | 108.99,76.81 108.99,72.69 R26.2 | 108.99,76.81 108.99,78.03 LED1.K | LED3.K 107.77,61.11 107.77,67.21 107.62,67.21 107.08,67.75 107.08,68.75 108.83,70.5 108.83,72.31 | 108.99,76.81 112.04,76.81 113.26,78.03 121.49,78.03 C6.- | JP19.1 133.99,10.06 137.34,10.06 JP20.1 137.8,10.06 138.1,10.36 138.1,20.27 C3.2 138.1,20.73 138.1,22.25 138.86,23.01 138.86,31.55 137.95,32.46 135.05,32.46 | R17.2 133.68,29.26 135.05,30.63 135.05,32.46 | 135.05,32.46 135.05,34.29 C13.2 135.05,34.59 135.05,39.32 C12.2 134.9,39.78 134.9,48.01 137.49,50.6 R20.2 | R23.2 129.87,64.62 v127.28,62.03 126.97,62.18 124.69,64.47 117.07,64.47 114.02,61.42 114.02,60.96 LED2.K 114.02,60.66 114.02,42.52 115.54,41 C8.- 115.54,40.54 115.54,35.2 114.48,34.14 114.48,32.61 115.85,31.24 SHUTTER_STEPPER.GND@0 116.15,30.79 116.15,30.33 117.22,29.26 117.22,17.37 116.15,16.31 SHUTTER_STEPPER.GND | 73.63,2.44 X3.24 71.81,4.12 61.14,4.12 58.85,6.4 58.55,6.55 | 80.19,10.52 PAN_STEPPER.GND 80.34,10.82 82.78,13.26 85.37,13.26 R7.2 85.67,13.11 92.68,13.11 94.97,10.82 95.58,10.82 PAN_STEPPER.GND@0 95.89,10.97 96.34,10.97 97.56,12.19 98.63,12.19 100.15,10.67 100.15,5.33 100.3,5.03 | 103.81,5.03 103.81,5.94 105.64,7.77 105.64,8.08 JP27.2 105.79,8.53 105.79,12.04 JP13.2 105.94,12.34 106.86,13.26 106.86,13.41 109.3,15.85 110.97,15.85 113.26,18.14 113.41,18.44 | 103.81,5.03 103.81,3.81 C7.- | 100.3,5.03 99.69,4.42 99.69,4.27 99.24,3.81 C2.- | 103.81,5.03 100.3,5.03 | 113.41,18.44 113.41,20.88 R11.2 | 113.41,18.44 115.85,16 SHUTTER_STEPPER.GND | JP17.2 115.54,12.5 115.54,15.7 SHUTTER_STEPPER.GND
  Bottom 0.813: U1.GND@2 27.91,76.2 29.29,77.57 43.31,77.57 48.18,72.69 52.91,72.69 55.04,70.56 JP18.2 55.04,70.1 55.04,66.14 JP32.2 55.04,65.68 62.2,58.52 ?_STEPPER.GND 65.1,60.96 R12.2 69.22,60.81 74.85,60.81 77.29,58.37 ?_STEPPER.GND@0 77.29,57.91 77.29,55.63 C9.- 76.83,55.32 73.02,55.32 70.89,53.19 62.66,53.19 56.87,47.4 56.87,39.47 55.04,37.64 55.04,37.34 | X3.19 52.45,2.29 48.79,2.29 X3.18 48.34,2.29 44.22,2.29 X3.17 44.37,2.59 44.37,7.47 X3.5 | C11.- 61.44,13.41 61.44,18.14 61.29,18.29 C14.2 | X3.5 44.22,7.92 47.88,11.58 47.88,12.65 JP28.2 48.18,11.43 51.69,7.92 52.45,7.92 X3.7 52.91,7.62 54.43,6.1 58.09,6.1 58.55,6.55 | 58.55,6.55 58.55,8.38 61.44,11.28 61.44,12.95 C11.- | U1.GND@0 41.48,27.89 37.82,24.23 37.82,23.01 C1.2 37.67,22.55 37.67,13.56 C10.- 37.36,13.26 37.36,9.6 | U1.GND@1 44.07,27.89 41.93,27.89 U1.GND@0 | 37.36,9.6 37.36,9.45 35.84,7.92 X3.3 | JP29.2 23.95,12.65 23.95,12.34 26.69,9.6 34.16,9.6 35.53,8.23 X3.3 | X3.15 35.84,2.44 35.84,7.47 X3.3 | 37.36,9.6 41.33,9.6 43.15,7.77 43.76,7.77 X3.5 | WS2801.2 9.78,6.1 8.56,7.32 8.56,17.68 9.47,18.59 9.78,18.59 I2C_LCD.2 10.24,18.75 11,18.75 14.05,21.79 14.05,30.18 C4.2 14.35,30.48 14.35,36.88 COLOUR_STEPPER.GND 15.27,37.64 17.55,39.93 21.21,39.93 R9.2 21.67,39.93 24.56,39.93 25.63,38.86 28.37,38.86 29.74,37.49 COLOUR_STEPPER.GND@0 | R10.2 67.54,39.93 65.1,39.93 62.66,37.49 GOBO_STEPPER.GND 62.2,37.34 60.83,35.97 56.41,35.97 55.04,37.34 | 55.04,37.34 54.43,37.34 TILT_STEPPER.GND@0 53.98,37.64 53.52,37.64 51.38,39.78 44.37,39.78 R8.2 44.07,39.93 41.63,39.93 39.19,37.49 TILT_STEPPER.GND
  Bottom 0.813: COLOUR_STEPPER.GND@0 30.05,37.34 30.05,31.55 28.98,30.48 C5.- | TILT_STEPPER.GND 38.73,37.64 34.47,37.64 33.25,38.86 31.72,38.86 30.5,37.64 COLOUR_STEPPER.GND@0 | TILT_STEPPER.GND 41.48,35.05 41.48,28.35 U1.GND@0 | 108.83,72.31 R26.2 | 108.83,72.31 106.04,72.31 C15.2 | v65.33,13.25 61.63,13.25 C11.-
GOBO_DIR
  Bottom 0.406: GOBO_STEPPER.DIR 62.66,50.14 63.12,49.68 63.12,49.53 70.13,42.52 86.44,42.52 94.82,50.9 U1.D40
GOBO_EN
  Top 0.406: R4.1 79.12,47.7 79.12,48.92 80.34,50.14 GOBO_STEPPER.EN
  Bottom 0.406: U1.D38 83.54,53.34 80.34,50.14 GOBO_STEPPER.EN
GOBO_STEP
  Bottom 0.406: GOBO_STEPPER.STEP 65.1,50.29 66.17,50.29 68.15,52.27 81.56,52.27 83.24,53.95 93.9,53.95 94.51,54.56 96.19,54.56 97.41,53.34 U1.D39
GOBO_STOP  (via drill 0.61)
  Top 0.406: v78.36,33.53 78.36,19.66 74.7,16 74.09,16 JP16.1
  Bottom 0.406: v78.36,33.53 94.36,49.53 95.43,49.53 96.65,50.75 97.41,50.75 U1.D41 | JP30.1 68.91,12.65 70.89,10.67 71.96,10.67 72.72,11.43 72.72,14.63 73.94,15.85 JP16.1
I2C_SCL  (via drill 0.6 pad 1.27)
  Top 0.406: v14.58,66.25 14.58,66.22 v9.93,61.57
  Bottom 0.406: I2C_LCD.4 9.93,22.71 9.93,55.75 v9.93,61.57 | U1.D21 87.2,76.2 84.3,79.1 26.09,79.1 23.65,76.66 23.65,75.29 23.62,75.29 v14.58,66.25
I2C_SDA
  Bottom 0.406: I2C_LCD.3 9.93,20.73 11.76,20.73 13.13,22.1 13.13,67.06 25.78,79.7 85.52,79.7 88.57,76.66 88.57,75.74 87.81,74.98 86.13,74.98 84.91,76.2 U1.D20
JTAG0
  Bottom 0.406: U1.A4 61.9,27.89 61.14,27.89 56.41,23.16 JTAG.1
JTAG2
  Bottom 0.406: U1.A6 66.93,27.89 66.17,27.89 61.44,23.16 JTAG.3
JTAG3
  Bottom 0.406: U1.A7 69.52,27.89 68.76,27.89 64.03,23.16 JTAG.4
N$1
  Top 0.406: PAN_STEPPER.SLP 85.52,23.47 87.96,23.47 PAN_STEPPER.RST
N$2
  Top 0.406: TILT_STEPPER.SLP 44.22,50.14 46.66,50.14 TILT_STEPPER.RST
N$3
  Top 0.406: COLOUR_STEPPER.SLP 20.14,50.14 22.43,50.14 COLOUR_STEPPER.RST
N$4
  Top 0.406: GOBO_STEPPER.SLP 67.69,50.14 70.13,50.14 GOBO_STEPPER.RST
N$5
  Top 0.406: SHUTTER_STEPPER.RST SHUTTER_STEPPER.SLP
N$6
  Top 0.406: ?_STEPPER.SLP 67.69,71.17 70.13,71.17 ?_STEPPER.RST
N$7
  Bottom 0.406: 94.36,22.25 88.87,22.25 87.66,21.03 85.52,21.03 R7.1 | 94.36,22.25 95.58,23.47 PAN_STEPPER.MS1 | JP1.6 95.58,20.88 94.36,22.1 94.36,22.25
N$8
  Top 0.406: PAN_STEPPER.MS3 90.55,23.47 90.55,17.22 JP1.2
N$9
  Top 0.406: PAN_STEPPER.MS2 92.99,23.47 92.99,17.22 JP1.4
N$10
  Bottom 0.406: 53.06,48.92 47.73,48.92 46.51,47.7 44.22,47.7 R8.1 | TILT_STEPPER.MS1 53.06,48.92 | JP2.6 54.28,43.89 54.28,47.55 53.06,48.77 53.06,48.92
N$11
  Top 0.406: TILT_STEPPER.MS3 49.25,50.14 49.25,43.89 JP2.2
N$12
  Top 0.406: TILT_STEPPER.MS2 51.84,50.14 51.84,43.89 JP2.4
N$13
  Bottom 0.406: 28.83,48.92 23.49,48.92 22.28,47.7 21.36,47.7 R9.1 | 28.83,48.92 30.05,50.14 COLOUR_STEPPER.MS1 | JP3.6 30.05,43.89 30.05,47.55 28.83,48.77 28.83,48.92
N$14
  Top 0.406: COLOUR_STEPPER.MS3 25.17,50.14 25.17,43.89 JP3.2
N$15
  Top 0.406: COLOUR_STEPPER.MS2 27.61,50.14 27.61,43.89 JP3.4
N$16
  Bottom 0.406: 76.53,48.92 71.2,48.92 69.98,47.7 67.69,47.7 R10.1 | 76.53,48.92 77.75,50.14 GOBO_STEPPER.MS1 | JP4.6 77.75,43.89 77.75,47.55 76.53,48.77 76.53,48.92
N$17
  Top 0.406: JP4.2 GOBO_STEPPER.MS3
N$18
  Top 0.406: GOBO_STEPPER.MS2 75.31,50.14 75.31,43.89 JP4.4
N$19
  Bottom 0.406: 104.42,29.87 104.42,24.54 105.64,23.32 105.64,21.03 R11.1 | 104.42,29.87 103.2,31.09 SHUTTER_STEPPER.MS1 | JP5.6 109.45,31.09 105.79,31.09 104.57,29.87 104.42,29.87
N$20
  Top 0.406: SHUTTER_STEPPER.MS3 103.2,26.06 109.45,26.06 JP5.2
N$21
  Top 0.406: SHUTTER_STEPPER.MS2 103.2,28.65 109.45,28.65 JP5.4
N$22
  Bottom 0.406: R12.1 71.2,68.58 72.57,69.95 76.68,69.95 | 76.68,69.95 77.75,71.02 ?_STEPPER.MS1 | JP6.6 78.97,64.77 78.97,67.51 76.68,69.8 76.68,69.95
N$23
  Top 0.406: ?_STEPPER.MS3 72.72,70.1 73.94,68.89 73.94,64.77 JP6.2
N$24
  Top 0.406: JP6.4 75.31,65.99 75.31,71.02 ?_STEPPER.MS2
N$25
  Top 0.813: PAN_STEPPER.2B 92.99,10.67 92.99,7.62 JP7.1 93.14,7.32 93.14,3.2 JP23.1
N$26
  Top 0.813: PAN_STEPPER.2A 90.55,10.67 90.55,7.62 JP7.2 90.55,7.32 90.55,3.2 JP23.2
N$27
  Top 0.813: PAN_STEPPER.1A JP7.3 JP23.3
N$28  (via drill 0.61)
  Top 0.406: v128.96,34.59 128.04,33.68 127.28,33.68 IC1.3 | v128.96,43.13 127.28,43.13 IC2.2
  Bottom 0.406: v128.96,43.13 v128.96,34.59
N$29
  Top 0.406: C12.1 132.31,39.32 132.31,38.41 131.24,37.34 131.24,34.44 128.04,31.24 127.28,31.24 IC1.1 127.13,30.94 126.36,30.18 126.36,21.79 122.86,18.29 122.86,16.92 R18.2
N$30  (via drill 0.61)
  Top 0.406: v117.37,2.74 103.2,2.74 101.98,3.96 101.98,4.42 96.8,9.6 95.12,9.6 94.21,10.52 94.21,11.28 93.45,12.04 85.06,12.04 84,10.97 84,10.21 83.39,9.6 51.69,9.6 49.86,7.77 49.86,6.55 47.27,3.96 v41.63,3.96
  Bottom 0.406: v117.37,2.74 123.32,8.69 123.32,13.56 121.64,15.24 121.64,20.27 122.86,21.49 122.86,24.69 R28.2 | v41.63,3.96 40.11,2.44 X3.16
N$31
  Top 0.813: PAN_STEPPER.1B 85.37,10.67 85.37,7.62 JP7.4 85.52,7.32 85.52,3.2 JP23.4
N$32
  Bottom 0.813: TILT_STEPPER.2B 51.69,37.34 51.69,29.87 50.32,28.5 50.32,24.54 51.69,23.16 51.69,22.86 JP8.1 51.84,22.55 51.84,19.05 JP24.1
N$33
  Bottom 0.813: TILT_STEPPER.2A 49.25,37.34 49.25,22.86 JP8.2 49.25,22.55 49.25,19.05 JP24.2
N$34
  Bottom 0.813: TILT_STEPPER.1A 46.81,37.34 46.81,29.87 48.18,28.5 48.18,24.54 46.81,23.16 46.81,22.86 JP8.3 46.81,22.55 46.81,19.05 JP24.3
N$35  (via drill 0.61)
  Top 0.813: v45.74,29.41 47.27,29.41 48.18,28.5 48.18,27.43 46.51,25.76 43.31,25.76 41.63,24.08 41.63,20.73 43.31,19.05 JP24.4 44.22,19.36 44.22,22.86 JP8.4
  Bottom 0.813: v45.74,29.41 44.22,30.94 44.22,37.34 TILT_STEPPER.1B
N$36
  Bottom 0.813: COLOUR_STEPPER.2B 27.61,37.34 27.61,31.85 27,31.24 27,23.47 27.61,22.86 JP9.1 27.76,22.55 27.76,19.05 JP26.1
N$37
  Bottom 0.813: COLOUR_STEPPER.2A 25.17,37.34 25.17,33.68 26.09,32.77 26.09,31.7 25.78,31.39 25.78,23.47 25.17,22.86 JP9.2 25.17,22.55 25.17,19.05 JP26.2
N$38
  Top 0.813: COLOUR_STEPPER.1A 22.43,37.34 22.43,32.31 21.82,31.7 21.82,23.47 22.43,22.86 JP9.3 22.58,22.55 22.58,19.05 JP26.3
N$39
  Top 0.813: COLOUR_STEPPER.1B 20.14,37.34 20.14,31.55 20.75,30.94 20.75,23.47 20.14,22.86 JP9.4 20.14,22.55 20.14,19.05 JP26.4
N$40
  Top 0.813: GOBO_STEPPER.2B 75.16,37.34 75.16,30.48 73.18,28.5 73.18,25.15 75.16,23.16 75.16,22.86 JP10.1 75.31,22.55 75.31,19.05 JP21.1
N$41  (via drill 0.61)
  Top 0.813: v72.72,30.02 GOBO_STEPPER.2A
  Bottom 0.813: v72.72,30.02 JP10.2 JP21.2
N$42
  Top 0.813: GOBO_STEPPER.1A 70.28,37.34 70.28,30.79 72.11,28.96 72.11,24.99 70.28,23.16 70.28,22.86 JP10.3 70.28,22.55 70.28,19.05 JP21.3
N$43
  Top 0.813: GOBO_STEPPER.1B 67.69,37.34 67.69,31.85 71.04,28.5 71.04,26.52 67.69,23.16 67.69,22.86 JP10.4 67.69,22.55 67.69,19.05 JP21.4
N$44
  Top 0.813: SHUTTER_STEPPER.2B 116,28.65 116,29.26 117.22,30.48 117.22,34.29 112.8,38.71 111.58,38.71 JP11.1 111.58,39.01 111.58,42.52 JP22.1
N$45
  Top 0.813: SHUTTER_STEPPER.2A 115.85,26.06 115.85,26.67 113.56,28.96 113.56,33.83 108.99,38.41 108.99,38.71 JP11.2 109.14,39.01 109.14,42.52 JP22.2
N$46
  Bottom 0.813: SHUTTER_STEPPER.1A 115.85,23.62 115.85,24.08 113.56,26.36 113.56,31.7 108.69,36.58 108.23,36.58 106.4,38.41 106.4,38.71 JP11.3 106.55,39.01 106.55,42.52 JP22.3
N$47  (via drill 0.61)
  Top 0.813: v108.08,30.18 108.08,34.29 103.96,38.41 103.96,38.71 JP11.4 103.96,39.01 103.96,42.52 JP22.4
  Bottom 0.813: v108.08,30.18 108.08,25.45 108.99,24.54 111.58,24.54 115.09,21.03 115.85,21.03 SHUTTER_STEPPER.1B
N$48
  Bottom 0.813: ?_STEPPER.2B 75.16,58.37 74.55,58.37 70.59,54.41 49.1,54.41 46.96,56.54 JP12.1 47.27,57 47.27,61.27 JP25.1
N$49
  Top 0.813: ?_STEPPER.2A 72.72,58.37 72.11,58.37 68.15,54.41 51.69,54.41 49.55,56.54 JP12.2 49.71,57 49.71,61.27 JP25.2
N$50
  Bottom 0.813: 54.28,59.13 55.04,59.13 57.17,57 68.15,57 69.52,58.37 70.13,58.37 ?_STEPPER.1A | 54.28,59.13 52.45,60.96 52.45,61.27 JP25.3 | JP12.3 52.3,56.69 52.3,57 54.13,58.83 54.28,59.13
N$51
  Top 0.813: ?_STEPPER.1B 67.54,58.37 66.93,58.37 65.25,56.69 54.74,56.69 JP12.4 54.89,57 54.89,61.27 JP25.4
N$52  (via drill 0.61)
  Top 0.406: v126.21,20.27 126.21,12.95 124.84,11.58 124.84,9.3 R13.1 | v117.53,63.25 117.53,65.38 111.58,71.32 111.58,78.03 LED1.A
  Bottom 0.406: v126.21,20.27 126.21,54.56 v117.53,63.25
N$53  (via drill 0.6 pad 1.27, 0.61)
  Top 0.406: v20.14,48.62 12.58,41.05 12.58,27.5 15.83,24.25 v15.83,12.75
  Bottom 0.406: v20.14,48.62 21.36,49.84 21.36,55.02 42.55,76.2 U1.D8 | WS2801.3 9.93,8.08 9.93,8.53 11.61,8.53 v15.83,12.75
N$54  (via drill 0.61)
  Top 0.406: v119.05,9.75 118.75,9.75 118.14,10.36 117.53,10.36 116.61,11.28 116.61,13.72 115.7,14.63 114.02,14.63 111.58,17.07 v110.52,17.07
  Bottom 0.406: v119.05,9.75 119.51,9.3 122.25,9.3 R13.2 | v110.52,17.07 106.1,17.07 103.66,14.63 97.26,14.63 96.04,15.85 79.58,15.85 73.02,9.3 62.51,9.3 61.14,7.92 X3.9
N$55
  Top 0.406: LED3.A 105.33,60.96 105.33,58.37 114.33,49.38 114.33,38.41 119.66,33.07 119.66,17.22 123.62,13.26 123.62,6.86 124.84,5.64 R15.2
N$56
  Bottom 0.406: LED2.A 116.61,60.96 116.61,57.3 125.3,48.62 125.3,13.56 124.84,13.11 R14.1
N$57  (via drill 0.6 pad 1.27)
  Top 0.406: v24.58,61.5 16.33,53.25 16.33,49.99 11.3,44.96 11.3,14.22 v10.83,13.75
  Bottom 0.406: 9.93,10.06 WS2801.4 10.83,10.96 v10.83,13.75 | U1.D9 39.28,76.2 v24.58,61.5
N$58
  Bottom 0.406: X3.11 70,7.83 72.33,5.5 78.33,5.5 83.33,0.5 139.08,0.5 140.08,1.5 140.08,73.25 130.33,83 107.08,83 103.83,79.75 103.83,56.52 F1.1
  Bottom 0.813: X3.10 65.25,7.77 69.37,7.77 X3.11
N$60  (via drill 0.6 pad 1.27)
  Top 0.813: 25.02,78.33 25.58,78.33 | 25.58,78.33 97.41,78.33 102.13,73.61 102.13,54.56 105.64,51.05 105.64,48.92 F2.1 | 25.58,78.33 25.5,78.25 13.08,78.25 3.33,68.5 3.33,5.5 7.58,1.25 16.08,1.25 20.58,5.75 v40.08,5.75 40.33,5.75 41.58,5.75 41.93,6.1 v46.66,6.1
  Bottom 0.813: X3.23 69.37,2.29 65.56,2.29 X3.22 65.1,2.29 61.14,2.29 X3.21 60.68,2.59 59.61,2.59 57.17,5.03 51.54,5.03 48.79,7.77 X3.6 48.34,7.77 v46.66,6.1 | X3.4 40.11,7.77 40.11,5.78 v40.08,5.75
N$61
  Top 0.406: 132.77,40.54 132,40.54 131.24,39.78 131.24,38.25 128.04,35.05 127.28,35.05 IC1.4 | 132.77,40.54 133.53,39.78 133.53,35.36 132.46,34.29 C13.1 | R21.2 137.49,45.41 132.77,40.69 132.77,40.54
N$62
  Top 0.406: IC5.3 127.13,55.32 125.45,55.32 124.54,56.24 124.54,63.4 126.52,65.38 127.13,65.38 IC6.2
N$63  (via drill 0.61)
  Top 0.406: v130.02,54.1 128.65,52.73 127.28,52.73 IC5.1 | v132.46,65.99 v132.46,56.54 | v95.27,30.94 v89.79,30.94
  Bottom 0.406: v132.46,56.54 v130.02,54.1 | v132.46,65.99 130.02,68.43 R24.2 129.87,68.73 129.57,69.04 116,69.04 112.8,65.84 112.8,52.58 105.18,44.96 105.18,33.98 103.66,32.46 102.89,32.46 101.37,30.94 v95.27,30.94 | v89.79,30.94 72.26,30.94 71.81,30.48 71.81,28.5 69.98,26.67 68.91,26.67 66.47,24.23 66.47,23.16 64.34,21.03 62.36,21.03 59.77,18.44 58.85,18.44 C14.1
N$64  (via drill 0.61)
  Top 0.406: v125.45,56.69 125.6,56.54 127.13,56.54 IC5.4 | v119.81,62.33 114.48,62.33 108.99,67.82 R27.2
  Bottom 0.406: v119.81,62.33 v125.45,56.69 | R27.2 108.99,67.82 108.99,60.66 108.23,59.89 107.31,59.89 106.7,60.5 106.7,66.88 106.08,67.5 106.08,69.58 C15.1
PAN_DIR  (via drill 0.61)
  Top 0.406: PAN_STEPPER.DIR 80.34,24.38 83.54,27.58 83.54,54.25 v84.15,54.86 | v89.94,56.54 89.94,67.67 v93.45,71.17
  Bottom 0.406: v84.15,54.86 88.27,54.86 v89.94,56.54 | v93.45,71.17 94.82,71.17 U1.D24
PAN_EN  (via drill 0.61)
  Top 0.406: R1.1 96.95,21.03 96.95,22.4 98.02,23.47 PAN_STEPPER.EN 98.02,23.62 96.19,25.45 96.19,46.18 96.95,46.94 97.87,46.94 100.3,49.38 v100.3,59.59
  Bottom 0.406: v100.3,59.59 101.22,60.5 101.22,66.6 98.02,69.8 97.1,69.8 96.19,70.71 96.19,71.63 94.97,72.85 94.97,73.61 U1.D22
PAN_ENCODER_A
  Top 0.406: R18.1 130.48,16.92 134.59,21.03 134.59,21.18 136.88,23.47 137.49,23.47 R16.2 136.88,23.62 133.68,26.82 R17.1
  Bottom 0.406: JP19.3 133.83,5.03 131.85,7.01 131.85,15.39 130.48,16.76 R18.1
PAN_ENCODER_B  (via drill 0.61)  (1 unrouted)
  Top 0.406: v131.39,33.22 131.7,32.92 131.7,22.86 130.63,21.79 130.63,19.96 R19.2
  Bottom 0.406: R20.1 R21.1 130.02,46.63 130.02,35.05 131.39,33.68 v131.39,33.22
PAN_ENCODER_CLK
  Top 0.406: IC1.6 127.13,37.49 126.52,37.49 125.75,38.25 125.75,43.74 126.36,44.35 127.13,44.35 IC2.3
PAN_STEP  (via drill 0.61)
  Top 0.406: v85.98,47.09 85.98,27.43 82.93,24.38 82.93,23.62 PAN_STEPPER.STEP | v89.03,50.14 89.03,69.49 v93.45,73.91
  Bottom 0.406: v89.03,50.14 v85.98,47.09 | v93.45,73.91 94.36,74.83 96.19,74.83 97.41,73.61 U1.D23
PAN_STOP  (via drill 0.61)
  Top 0.406: v100.3,65.84 100.3,60.96 101.22,60.05 101.22,26.36 102.89,24.69 103.66,24.69 109.6,18.75 109.6,16.61 111.73,14.48 113.26,14.48 114.17,13.56 114.17,9.6 114.02,9.45 114.02,7.01 113.11,6.1 105.18,6.1 103.2,8.08 JP27.1 JP13.1
  Bottom 0.406: v100.3,65.84 97.56,68.58 U1.D27
PS_ON
  Top 0.406: R28.1 130.48,24.69 130.48,22.55 127.89,19.96 127.89,7.01 129.87,5.03 PSON.2
SHUTTER_DIR
  Bottom 0.406: SHUTTER_STEPPER.DIR 103.2,16.76 96.8,23.16 96.8,28.04 91.01,33.83 91.01,45.26 91.47,45.72 U1.D44
SHUTTER_EN
  Top 0.406: R5.1 105.64,32.46 104.27,32.46 103.2,33.53 SHUTTER_STEPPER.EN
  Bottom 0.406: SHUTTER_STEPPER.EN 103.2,34.14 98.02,39.32 97.1,39.32 96.19,40.23 96.19,46.18 94.97,47.4 94.97,48.16 U1.D42
SHUTTER_STEP  (via drill 0.61)
  Top 0.406: v99.08,44.35 99.24,44.2 99.24,22.4 103.2,18.44 SHUTTER_STEPPER.STEP
  Bottom 0.406: v99.08,44.35 100,45.26 100,46.18 98.02,48.16 97.56,48.16 U1.D43
SHUTTER_STOP  (via drill 0.61)
  Top 0.406: v99.08,45.72 100.61,44.2 100.61,21.95 102.89,19.66 105.64,19.66 112.8,12.5 JP17.1 112.8,12.34 112.8,8.23 JP31.1
  Bottom 0.406: v99.08,45.72 U1.D45
TILT_DIR  (via drill 0.61)
  Top 0.406: v96.19,62.64 96.19,74.07 95.43,74.83 53.36,74.83 31.57,53.03 31.57,49.99 30.35,48.77 30.35,47.09 30.96,46.48 31.88,46.48 35.53,50.14 39.04,50.14 TILT_STEPPER.DIR
  Bottom 0.406: v96.19,62.64 95.73,62.64 94.97,63.4 U1.D30
TILT_EN  (via drill 0.61)
  Top 0.406: R2.1 55.65,47.7 55.65,49.07 56.72,50.14 TILT_STEPPER.EN 57.02,50.14 58.24,51.36 77.9,51.36 79.43,52.88 79.43,53.8 79.12,54.1 v79.12,57.3
  Bottom 0.406: v79.12,57.3 79.12,58.83 86.28,65.99 94.82,65.99 U1.D28
TILT_ENCODER_A  (via drill 0.61)
  Top 0.406: R24.1 137.64,68.43 137.64,64.92 R23.1 137.49,64.62 R22.2 137.64,60.2 138.56,59.28 138.56,23.01 137.03,21.49 137.03,20.12 v130.94,14.02
  Bottom 0.406: v130.94,14.02 127.89,10.97 127.89,7.01 128.65,6.25 131.09,6.25 131.85,5.49 131.85,4.57 132.77,3.66 135.2,3.66 136.42,4.88 137.64,4.88 JP20.3
TILT_ENCODER_B  (via drill 0.61)
  Top 0.406: R27.1 116.61,67.97 116.61,72.39 R26.1 | v127.28,27.58 127.28,5.03 128.65,3.66 131.09,3.66 131.85,4.42 131.85,5.33 132.77,6.25 135.2,6.25 136.42,7.47 137.64,7.47 JP20.2
  Bottom 0.406: R27.1 116.61,67.82 128.5,67.82 131.09,65.23 131.09,65.08 137.49,58.67 R25.2 137.34,55.78 133.83,52.27 133.83,34.14 v127.28,27.58
TILT_ENCODER_CLK
  Top 0.406: IC5.6 127.28,59.13 128.04,59.13 128.65,59.74 128.65,65.99 128.04,66.6 127.28,66.6 IC6.3
TILT_STEP  (via drill 0.6 pad 1.27)
  Top 0.406: v41.58,54.25 41.58,62.13 52.3,72.85 52.68,72.85 54.08,74.25 v85.33,74.25
  Bottom 0.406: 93.58,69.8 95.43,69.8 96.19,69.04 96.19,67.36 97.41,66.14 U1.D29 | 93.58,69.8 93.45,69.8 | TILT_STEPPER.STEP 41.63,50.29 41.63,54.2 v41.58,54.25 | v85.33,74.25 89.13,74.25 93.58,69.8
TILT_STOP  (via drill 0.61)
  Top 0.406: v98.48,59.74 97.1,59.74 96.19,58.83 96.19,57.91 95.43,57.15 94.51,57.15 89.94,52.58 v89.94,52.43 | v59.46,38.25 59.46,32.31 55.5,28.35 55.5,24.84 54.28,23.62 54.28,19.05 51.23,16 50.62,16 JP14.1 50.47,16 50.47,24.08 49.71,24.84 43.61,24.84 42.85,24.08 v42.85,21.18
  Bottom 0.406: v98.48,59.74 97.56,60.66 97.56,60.96 U1.D33 | v89.94,52.43 84.3,52.43 80.8,48.92 79.88,48.92 78.97,49.84 78.97,50.6 78.21,51.36 69.67,51.36 68.76,50.44 68.76,49.68 68,48.92 64.64,48.92 63.73,49.84 63.73,50.6 62.97,51.36 62.05,51.36 59.46,48.77 v59.46,38.25 | v42.85,21.18 42.85,16 45.29,13.56 45.29,12.8 JP28.1
VCC  (via drill 0.61)
  Top 0.813: R6.2 72.72,65.53 72.57,65.38 72.57,63.7 73.94,62.33 JP6.1 74.4,62.18 76.53,62.18 JP6.3 76.83,62.18 78.97,62.18 JP6.5 | JP18.3 52.45,70.41 52.45,66.45 JP32.3 52.3,65.99 54.43,63.86 59,63.86 64.34,58.52 65.1,58.52 ?_STEPPER.VDD 64.95,58.83 v68.45,62.33 | JP16.3 68.91,15.85 53.67,15.85 50.77,12.95 JP28.3 50.47,12.65 49.4,11.58 49.4,11.43 48.49,10.52 44.83,10.52 43.92,11.43 43.92,14.48 45.29,15.85 JP14.3 44.68,15.7 40.11,20.27 40.11,28.8 39.34,29.57 v39.04,29.41 39.04,34.9 | 71.35,42.67 71.35,47.55 R4.2 | 71.35,42.67 72.72,41.3 JP4.1 73.02,41.3 75.16,41.3 JP4.3 75.62,41.3 77.75,41.3 JP4.5 | 65.1,39.32 GOBO_STEPPER.VDD | 65.1,39.32 68.3,42.52 71.04,42.52 71.35,42.67 | 23.65,42.67 23.65,44.35 23.8,44.5 23.8,47.55 R3.2 | 23.65,42.67 25.02,41.3 JP3.1 25.48,41.3 27.61,41.3 JP3.3 27.91,41.3 30.05,41.3 JP3.5 30.5,41.15 32.64,41.15 38.73,35.05 39.04,34.9 | COLOUR_STEPPER.VDD 17.55,37.49 17.55,38.1 21.97,42.52 23.34,42.52 23.65,42.67 | 47.73,42.67 47.73,44.2 47.88,44.35 47.88,47.55 R2.2 | 47.73,42.67 49.1,41.3 JP2.1 49.55,41.3 51.69,41.3 JP2.3 52.15,41.3 54.28,41.3 JP2.5 56.11,39.47 64.8,39.47 65.1,39.32 | 47.73,42.67 47.42,42.52 44.83,42.52 41.63,39.32 41.63,37.49 TILT_STEPPER.VDD 39.04,34.9 | 122.4,41.91 IC2.14 | 126.14,45.64 126.21,45.72 IC2.4 127.58,45.57 128.35,45.57 130.18,43.74 130.18,42.67 129.41,41.91 IC2.1 | 126.14,45.64 122.4,41.91 | 126.21,32.31 125.15,31.24 121.18,31.24 IC1.14 121.34,30.79 121.34,24.69 122.86,23.16 122.86,19.96 R19.1 | 126.21,32.31 127.13,32.31 IC1.2 | 126.21,36.12 127.13,36.12 IC1.5 | 126.21,36.12 125.6,35.51 125.6,33.07 126.06,32.61 126.21,32.31
  Top 0.813: 122.4,41.91 122.55,41.6 122.55,39.93 126.06,36.42 126.21,36.12 | 122.4,64.16 121.18,64.16 IC6.14 | 126.06,67.82 122.4,64.16 | 126.06,67.82 127.13,67.82 IC6.4 | v126.67,73.46 125.6,72.39 125.6,68.43 125.91,68.12 126.06,67.82 | 124.99,52.73 122.71,52.73 | 122.71,52.73 121.18,52.73 IC5.14 120.73,52.58 117.07,48.92 116,48.92 F2.2 | 124.99,52.73 126.21,53.95 127.13,53.95 IC5.2 127.58,54.1 128.35,54.1 129.87,55.63 R25.1 129.87,56.08 128.19,57.76 | 128.19,57.76 127.28,57.76 IC5.5 126.82,57.76 126.21,57.76 125.6,58.37 125.6,62.03 127.13,63.55 127.13,64.01 IC6.1 | R22.1 129.87,59.28 128.5,57.91 128.19,57.76 | 122.71,52.73 122.71,60.96 122.55,61.11 122.55,63.86 122.4,64.16 | 126.14,45.64 125.15,46.63 125.15,52.43 124.99,52.73 | JP20.4 137.64,2.44 133.99,2.44 JP19.4 133.53,2.44 130.18,2.44 PSON.1 129.87,2.44 126.06,2.44 123.01,5.49 122.4,5.49 R15.1 | 89.03,16 89.03,17.68 89.18,17.83 89.18,20.88 R1.2 | 89.03,16 90.4,14.63 JP1.1 90.86,14.63 92.99,14.63 JP1.3 93.45,14.63 95.58,14.63 JP1.5 95.89,14.48 106.1,14.48 108.23,12.34 JP13.3 108.38,12.04 108.38,8.23 JP27.3 | 82.93,12.65 82.93,10.82 PAN_STEPPER.VDD | 82.93,12.65 86.13,15.85 88.72,15.85 89.03,16 | 82.93,12.65 74.09,12.65 JP30.3 | 110.67,24.54 109.14,24.54 108.99,24.69 105.79,24.69 R5.2 | 110.67,24.54 112.04,25.91 JP5.1 112.19,26.36 112.19,28.5 JP5.3 112.19,28.96 112.19,31.09 JP5.5 | JP17.3 117.83,12.5 117.83,15.85 116,17.68 116,18.29 SHUTTER_STEPPER.VDD 115.54,18.59 113.87,18.59 110.82,21.64 110.82,24.23 110.67,24.54
  Bottom 0.813: v68.45,62.33 73.94,62.33 JP6.1 | WS2801.1 9.93,4.12 12.67,4.12 21.21,12.65 JP29.3 | I2C_LCD.1 9.93,16.61 17.37,16.61 JP29.3 | JP29.3 21.21,13.11 21.21,15.85 JP15.3 20.9,16 20.29,16 17.55,18.75 17.55,37.34 COLOUR_STEPPER.VDD | C1.1 35.38,23.01 35.38,24.23 39.04,27.89 U1.5V@0 39.04,28.35 v39.04,29.41 | JP3.5 34.16,45.26 34.16,51.05 49.1,65.99 52.3,65.99 JP32.3 | v126.67,73.46 126.67,78.03 C6.+ | R16.1 137.49,31.09 135.66,29.26 135.66,20.42 C3.1 135.2,20.12 132.61,20.12 130.63,18.14 129.87,18.14 126.21,14.48 126.21,8.84 123.01,5.64 122.4,5.64 R15.1 121.94,5.49 117.98,1.52 116.92,1.52 116,2.44 116,5.64 115.85,5.94 | 115.85,5.94 112.19,5.94 110.06,8.08 108.38,8.08 JP27.3 | 115.85,5.94 117.68,7.77 JP31.3 117.83,8.23 117.83,12.34 JP17.3 118.14,12.8 118.29,12.95 118.29,21.95 122.55,26.21 123.47,26.21 124.38,25.3 124.38,21.79 123.01,20.42 123.01,19.96 R19.1 | JP30.3 76.68,15.39 76.68,21.79 79.73,24.84 91.31,24.84 93.9,27.43 93.9,28.5 90.25,32.16 71.04,32.16 65.86,37.34 65.1,37.34 GOBO_STEPPER.VDD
